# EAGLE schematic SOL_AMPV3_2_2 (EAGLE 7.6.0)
C_RIGHT: (C) 2016, 2017 Universiteit Antwerpen; D_NAME: W. Beaumont; PROJECT_NAME: SOLID AMPLIFIER; S_REV: 2.2

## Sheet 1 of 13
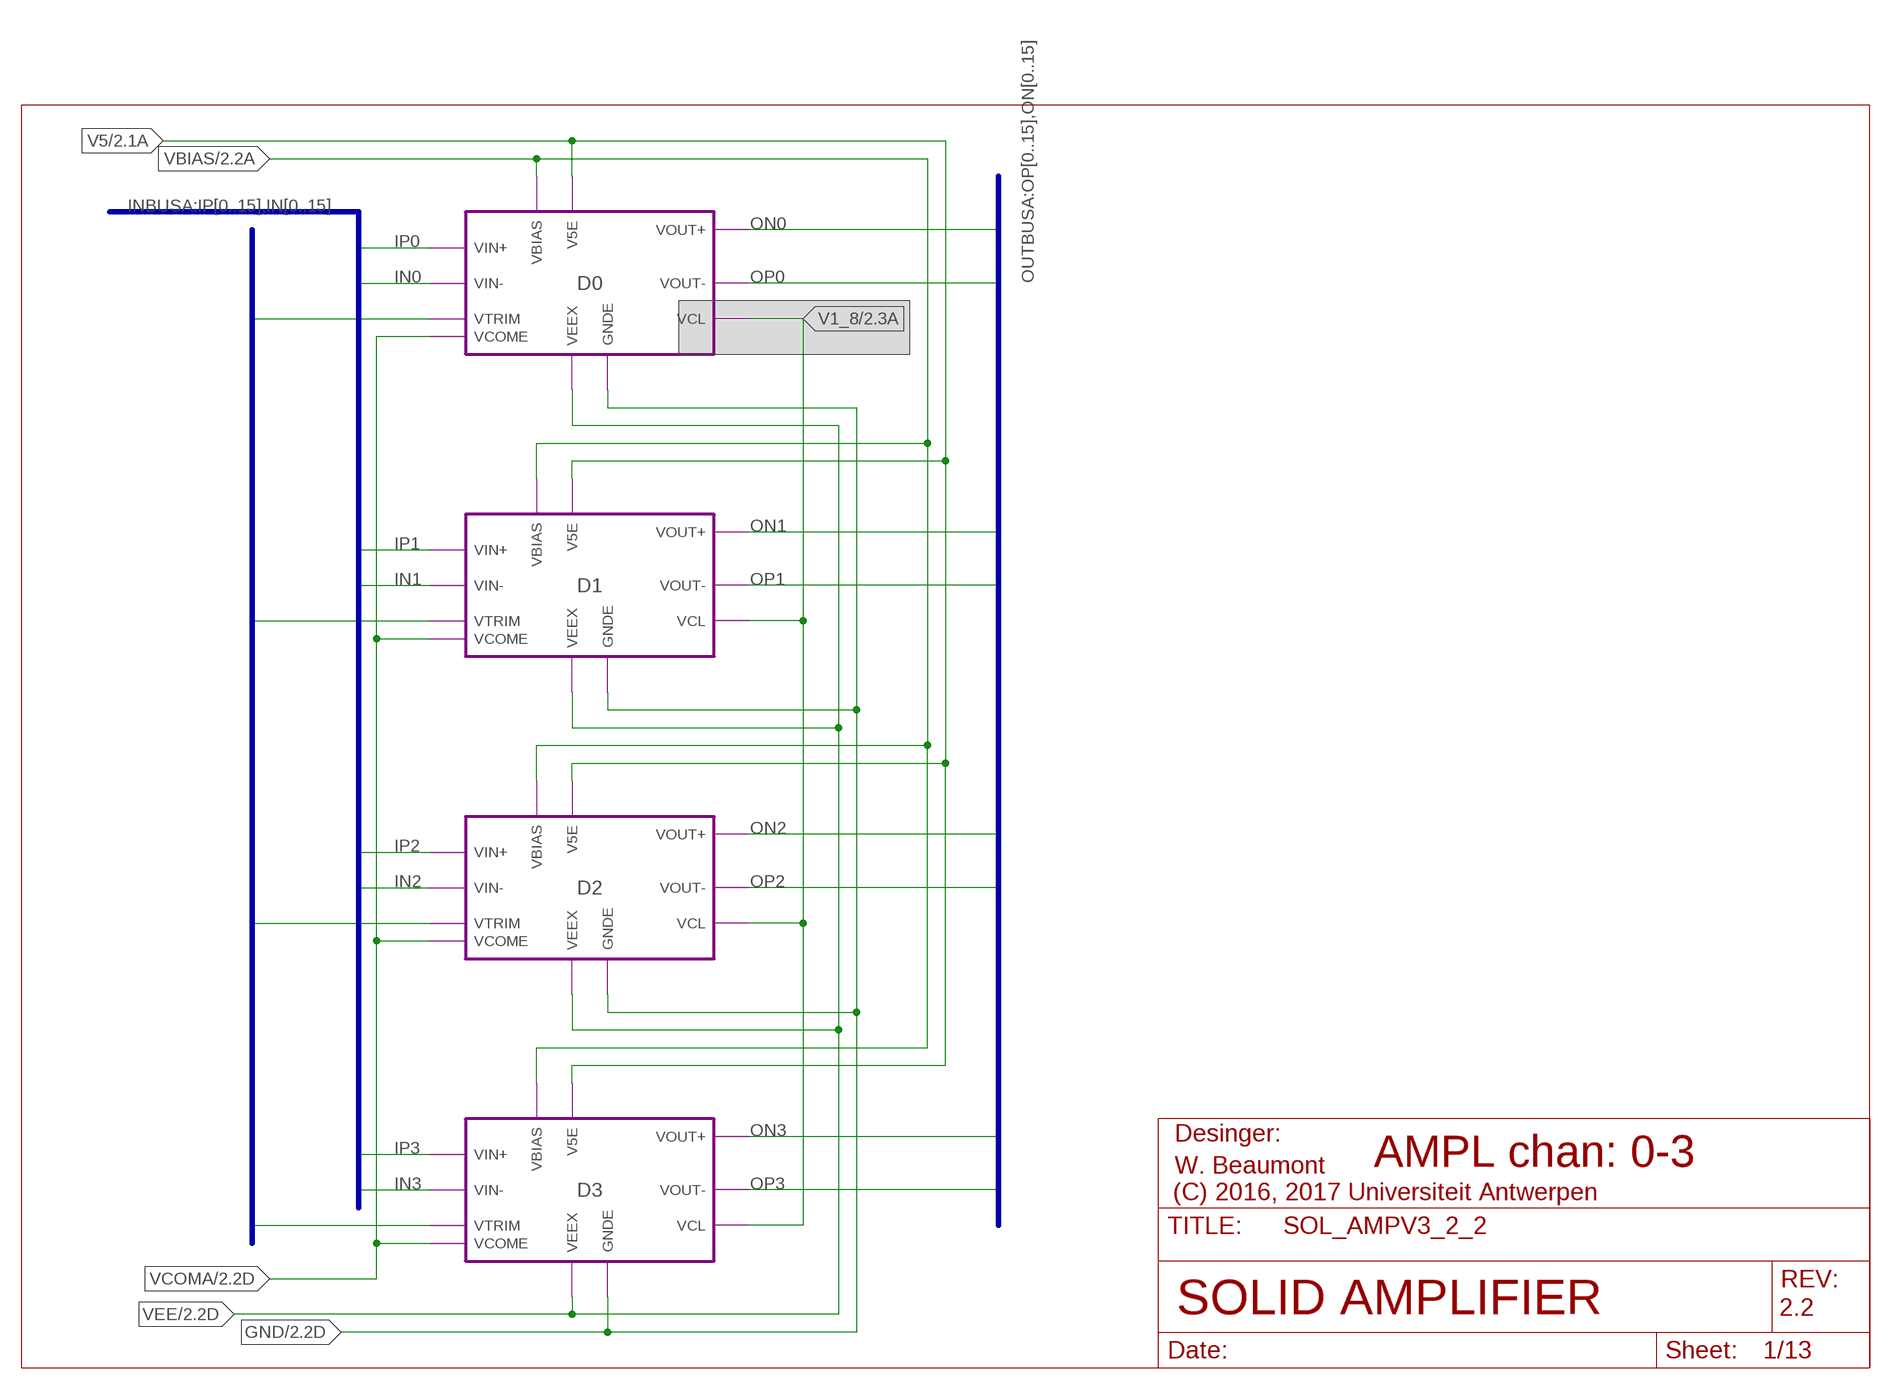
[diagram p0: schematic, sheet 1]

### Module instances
D0 = DIFFAMP$B
D1 = DIFFAMP$B
D2 = DIFFAMP$B
D3 = DIFFAMP$B

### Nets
GND: port D0.GNDE D1.GNDE D2.GNDE D3.GNDE ; also sheet 2,3,4,5,6,7,8,9,10,11,12,13
IN0: port D0.VIN- ; also sheet 5
IN1: port D1.VIN- ; also sheet 5
IN2: port D2.VIN- ; also sheet 5
IN3: port D3.VIN- ; also sheet 5
IP0: port D0.VIN+ ; also sheet 5
IP1: port D1.VIN+ ; also sheet 5
IP2: port D2.VIN+ ; also sheet 5
IP3: port D3.VIN+ ; also sheet 5
ON0: port D0.VOUT+ ; also sheet 5
ON1: port D1.VOUT+ ; also sheet 5
ON2: port D2.VOUT+ ; also sheet 5
ON3: port D3.VOUT+ ; also sheet 5
OP0: port D0.VOUT- ; also sheet 5
OP1: port D1.VOUT- ; also sheet 5
OP2: port D2.VOUT- ; also sheet 5
OP3: port D3.VOUT- ; also sheet 5
V1_8: port D3.VCL D0.VCL D1.VCL D2.VCL ; also sheet 2,3,4,5,6,7,8,9,10
V5: port D0.V5E D1.V5E D2.V5E D3.V5E ; also sheet 2,3,4,5,6,7,8,9,10,12,13
VBIAS [HV]: port D0.VBIAS D1.VBIAS D3.VBIAS D2.VBIAS ; also sheet 2,3,4,6,7,8,9,13
VCOMA: port D0.VCOME D3.VCOME D2.VCOME D1.VCOME ; also sheet 2,3,4,5
VEE: port D0.VEEX D1.VEEX D2.VEEX D3.VEEX ; also sheet 2,3,4,6,7,8,9,12
VTR0: port D0.VTRIM ; also sheet 11
VTR1: port D1.VTRIM ; also sheet 11
VTR2: port D2.VTRIM ; also sheet 11
VTR3: port D3.VTRIM ; also sheet 11

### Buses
OUTBUSA:OP[0..15],ON[0..15]
INBUSA:IP[0..15],IN[0..15]
VTRB:VTR[0..31]

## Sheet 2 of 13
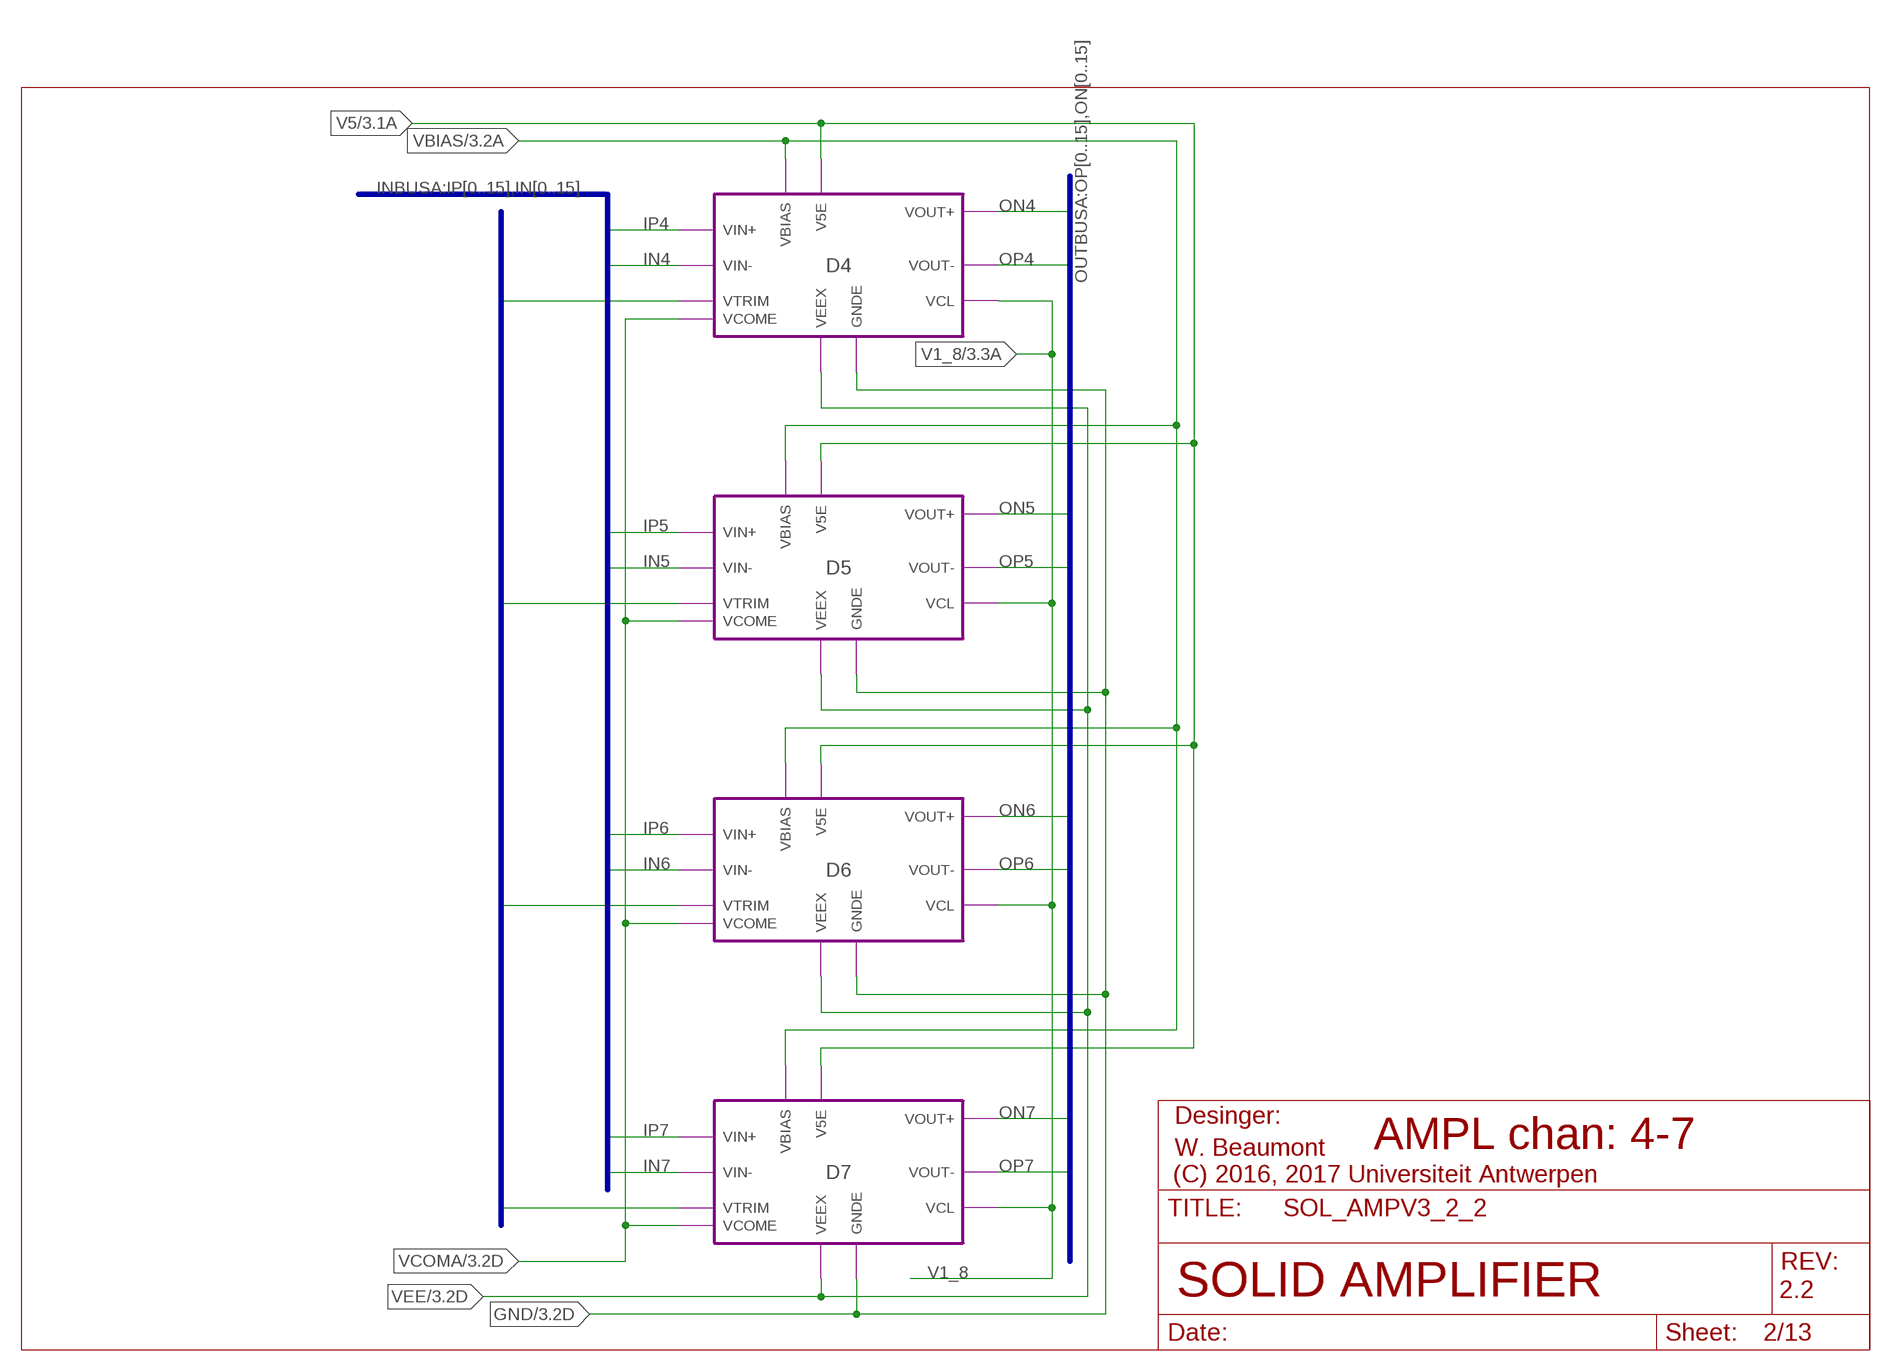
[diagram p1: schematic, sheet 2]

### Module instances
D4 = DIFFAMP$B
D5 = DIFFAMP$B
D6 = DIFFAMP$B
D7 = DIFFAMP$B

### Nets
GND: port D4.GNDE D5.GNDE D6.GNDE D7.GNDE ; also sheet 1,3,4,5,6,7,8,9,10,11,12,13
IN4: port D4.VIN- ; also sheet 5
IN5: port D5.VIN- ; also sheet 5
IN6: port D6.VIN- ; also sheet 5
IN7: port D7.VIN- ; also sheet 5
IP4: port D4.VIN+ ; also sheet 5
IP5: port D5.VIN+ ; also sheet 5
IP6: port D6.VIN+ ; also sheet 5
IP7: port D7.VIN+ ; also sheet 5
ON4: port D4.VOUT+ ; also sheet 5
ON5: port D5.VOUT+ ; also sheet 5
ON6: port D6.VOUT+ ; also sheet 5
ON7: port D7.VOUT+ ; also sheet 5
OP4: port D4.VOUT- ; also sheet 5
OP5: port D5.VOUT- ; also sheet 5
OP6: port D6.VOUT- ; also sheet 5
OP7: port D7.VOUT- ; also sheet 5
V1_8: port D4.VCL D7.VCL D6.VCL D5.VCL ; also sheet 1,3,4,5,6,7,8,9,10
V5: port D4.V5E D5.V5E D6.V5E D7.V5E ; also sheet 1,3,4,5,6,7,8,9,10,12,13
VBIAS [HV]: port D4.VBIAS D5.VBIAS D7.VBIAS D6.VBIAS ; also sheet 1,3,4,6,7,8,9,13
VCOMA: port D4.VCOME D7.VCOME D6.VCOME D5.VCOME ; also sheet 1,3,4,5
VEE: port D4.VEEX D5.VEEX D6.VEEX D7.VEEX ; also sheet 1,3,4,6,7,8,9,12
VTR4: port D4.VTRIM ; also sheet 11
VTR5: port D5.VTRIM ; also sheet 11
VTR6: port D6.VTRIM ; also sheet 11
VTR7: port D7.VTRIM ; also sheet 11

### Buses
OUTBUSA:OP[0..15],ON[0..15]
INBUSA:IP[0..15],IN[0..15]
VTRB:VTR[0..31]

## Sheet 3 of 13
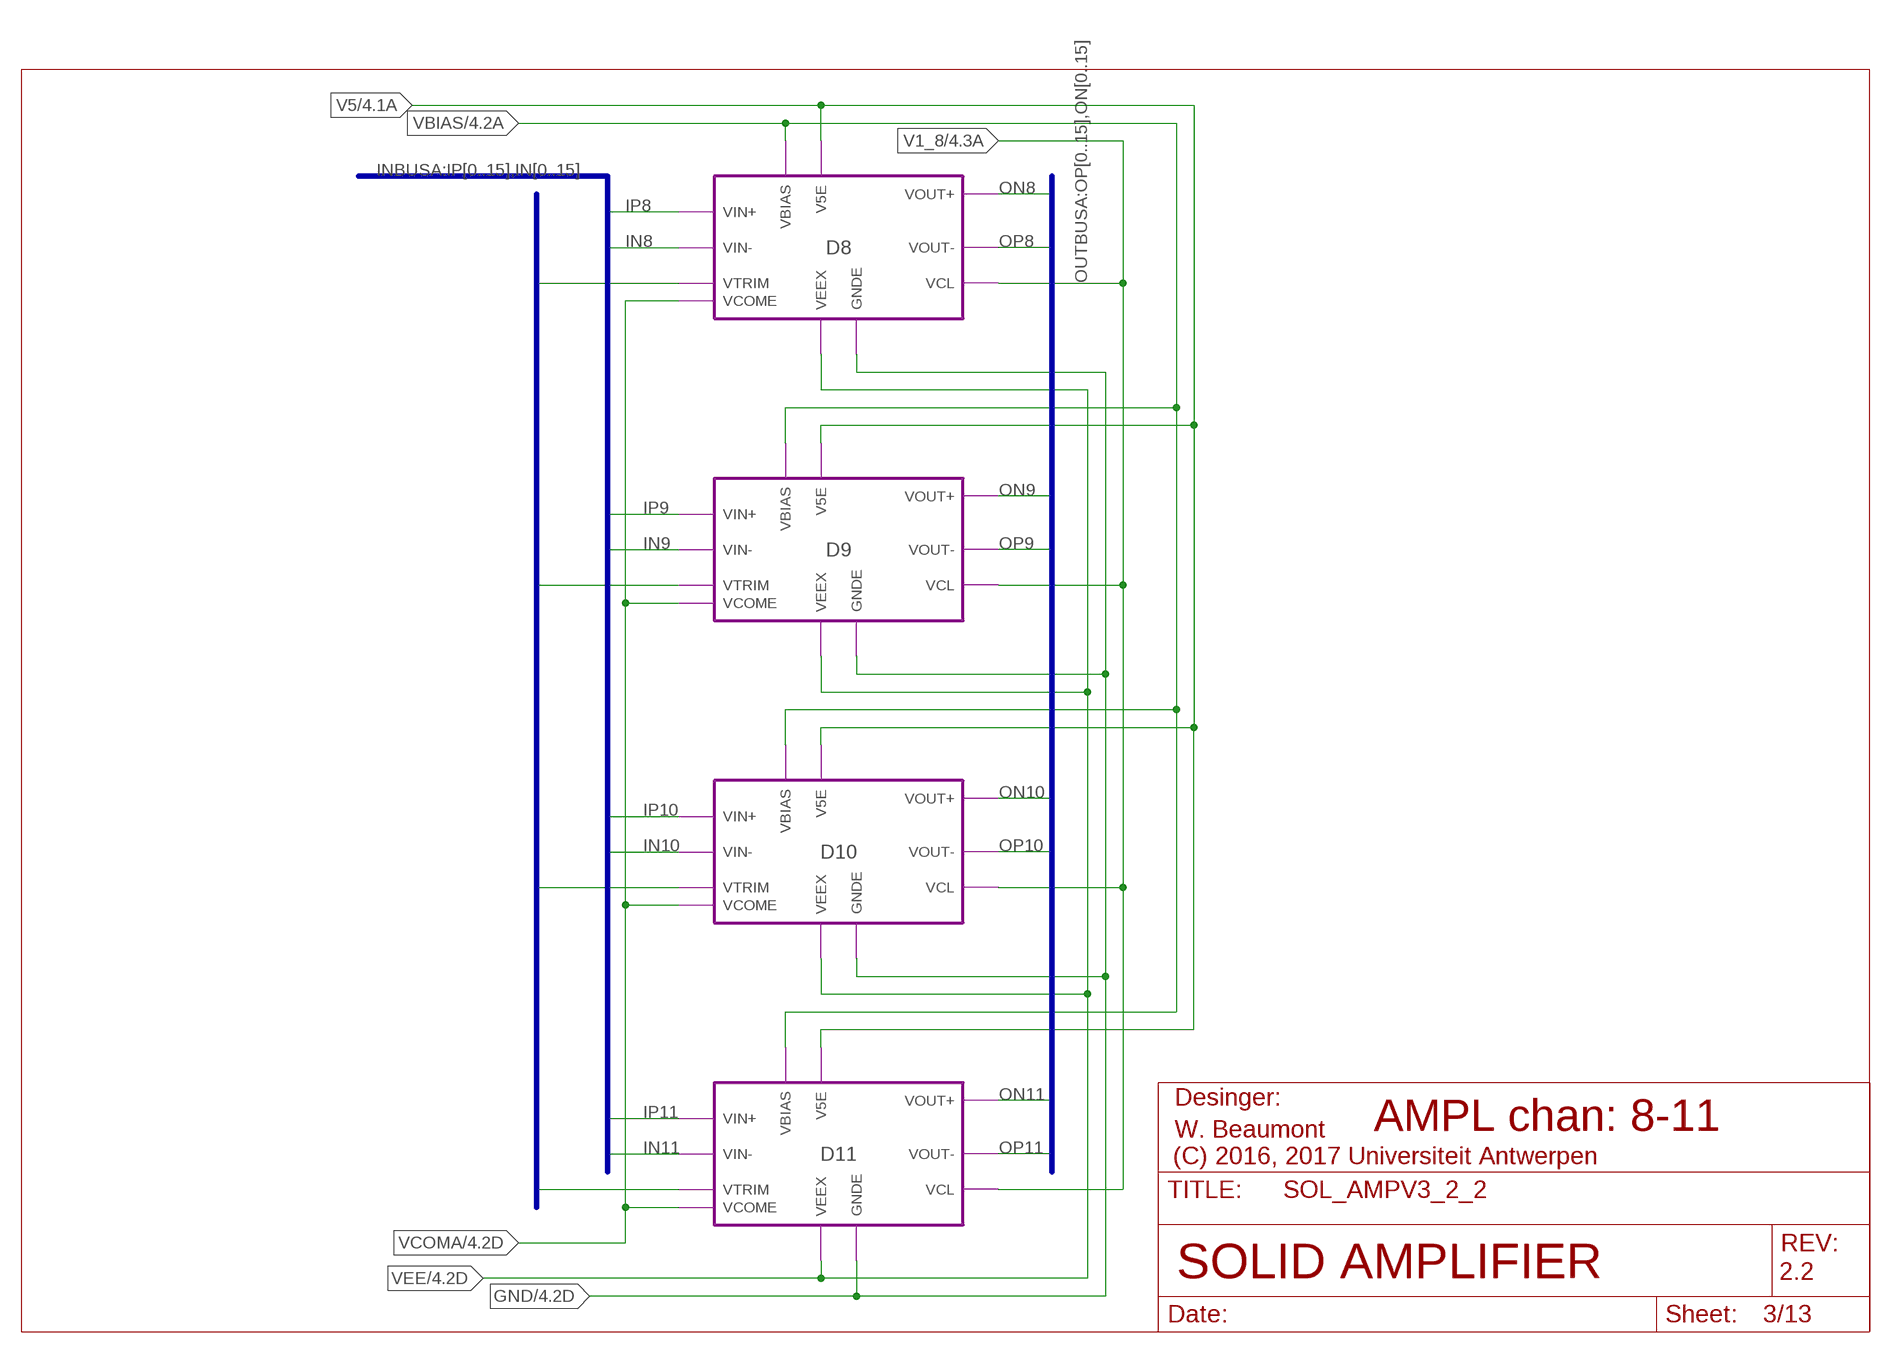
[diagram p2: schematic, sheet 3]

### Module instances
D8 = DIFFAMP$B
D9 = DIFFAMP$B
D10 = DIFFAMP$B
D11 = DIFFAMP$B

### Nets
GND: port D8.GNDE D9.GNDE D10.GNDE D11.GNDE ; also sheet 1,2,4,5,6,7,8,9,10,11,12,13
IN8: port D8.VIN- ; also sheet 5
IN9: port D9.VIN- ; also sheet 5
IN10: port D10.VIN- ; also sheet 5
IN11: port D11.VIN- ; also sheet 5
IP8: port D8.VIN+ ; also sheet 5
IP9: port D9.VIN+ ; also sheet 5
IP10: port D10.VIN+ ; also sheet 5
IP11: port D11.VIN+ ; also sheet 5
ON8: port D8.VOUT+ ; also sheet 5
ON9: port D9.VOUT+ ; also sheet 5
ON10: port D10.VOUT+ ; also sheet 5
ON11: port D11.VOUT+ ; also sheet 5
OP8: port D8.VOUT- ; also sheet 5
OP9: port D9.VOUT- ; also sheet 5
OP10: port D10.VOUT- ; also sheet 5
OP11: port D11.VOUT- ; also sheet 5
V1_8: port D11.VCL D10.VCL D9.VCL D8.VCL ; also sheet 1,2,4,5,6,7,8,9,10
V5: port D8.V5E D9.V5E D10.V5E D11.V5E ; also sheet 1,2,4,5,6,7,8,9,10,12,13
VBIAS [HV]: port D8.VBIAS D9.VBIAS D11.VBIAS D10.VBIAS ; also sheet 1,2,4,6,7,8,9,13
VCOMA: port D8.VCOME D11.VCOME D10.VCOME D9.VCOME ; also sheet 1,2,4,5
VEE: port D8.VEEX D9.VEEX D10.VEEX D11.VEEX ; also sheet 1,2,4,6,7,8,9,12
VTR8: port D8.VTRIM ; also sheet 11
VTR9: port D9.VTRIM ; also sheet 11
VTR10: port D10.VTRIM ; also sheet 11
VTR11: port D11.VTRIM ; also sheet 11

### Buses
OUTBUSA:OP[0..15],ON[0..15]
INBUSA:IP[0..15],IN[0..15]
VTRB:VTR[0..31]

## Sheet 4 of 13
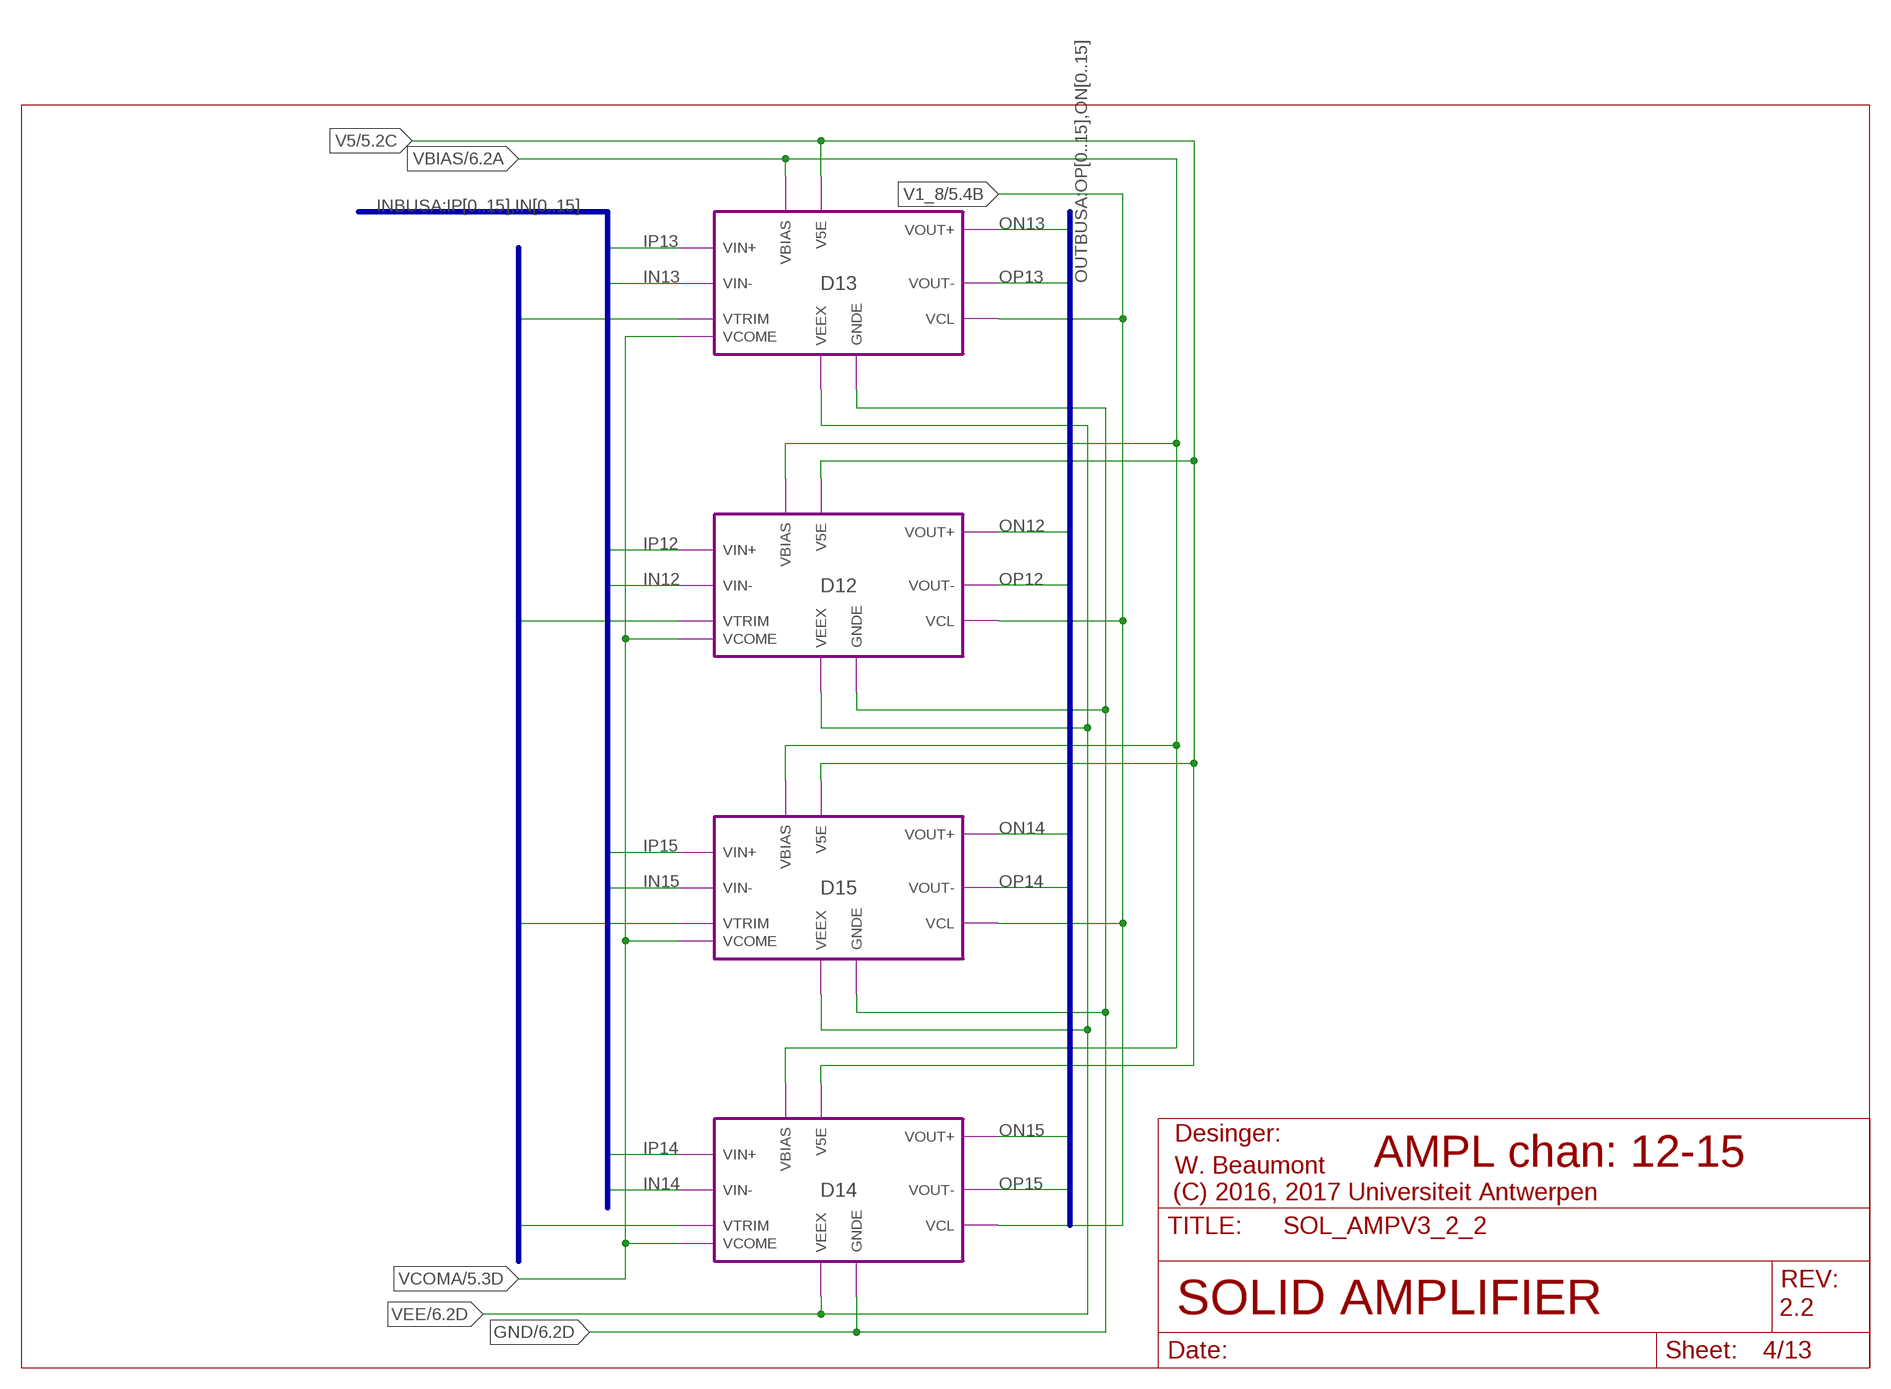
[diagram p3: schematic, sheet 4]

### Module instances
D13 = DIFFAMP$B
D12 = DIFFAMP$B
D15 = DIFFAMP$B
D14 = DIFFAMP$B

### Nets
GND: port D13.GNDE D12.GNDE D15.GNDE D14.GNDE ; also sheet 1,2,3,5,6,7,8,9,10,11,12,13
IN12: port D12.VIN- ; also sheet 5
IN13: port D13.VIN- ; also sheet 5
IN14: port D14.VIN- ; also sheet 5
IN15: port D15.VIN- ; also sheet 5
IP12: port D12.VIN+ ; also sheet 5
IP13: port D13.VIN+ ; also sheet 5
IP14: port D14.VIN+ ; also sheet 5
IP15: port D15.VIN+ ; also sheet 5
ON12: port D12.VOUT+ ; also sheet 5
ON13: port D13.VOUT+ ; also sheet 5
ON14: port D15.VOUT+ ; also sheet 5
ON15: port D14.VOUT+ ; also sheet 5
OP12: port D12.VOUT- ; also sheet 5
OP13: port D13.VOUT- ; also sheet 5
OP14: port D15.VOUT- ; also sheet 5
OP15: port D14.VOUT- ; also sheet 5
V1_8: port D13.VCL D12.VCL D15.VCL D14.VCL ; also sheet 1,2,3,5,6,7,8,9,10
V5: port D13.V5E D12.V5E D15.V5E D14.V5E ; also sheet 1,2,3,5,6,7,8,9,10,12,13
VBIAS [HV]: port D13.VBIAS D12.VBIAS D14.VBIAS D15.VBIAS ; also sheet 1,2,3,6,7,8,9,13
VCOMA: port D13.VCOME D14.VCOME D15.VCOME D12.VCOME ; also sheet 1,2,3,5
VEE: port D13.VEEX D12.VEEX D15.VEEX D14.VEEX ; also sheet 1,2,3,6,7,8,9,12
VTR12: port D13.VTRIM ; also sheet 11
VTR13: port D12.VTRIM ; also sheet 11
VTR14: port D15.VTRIM ; also sheet 11
VTR15: port D14.VTRIM ; also sheet 11

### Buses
OUTBUSA:OP[0..15],ON[0..15]
INBUSA:IP[0..15],IN[0..15]
VTRB:VTR[0..31]

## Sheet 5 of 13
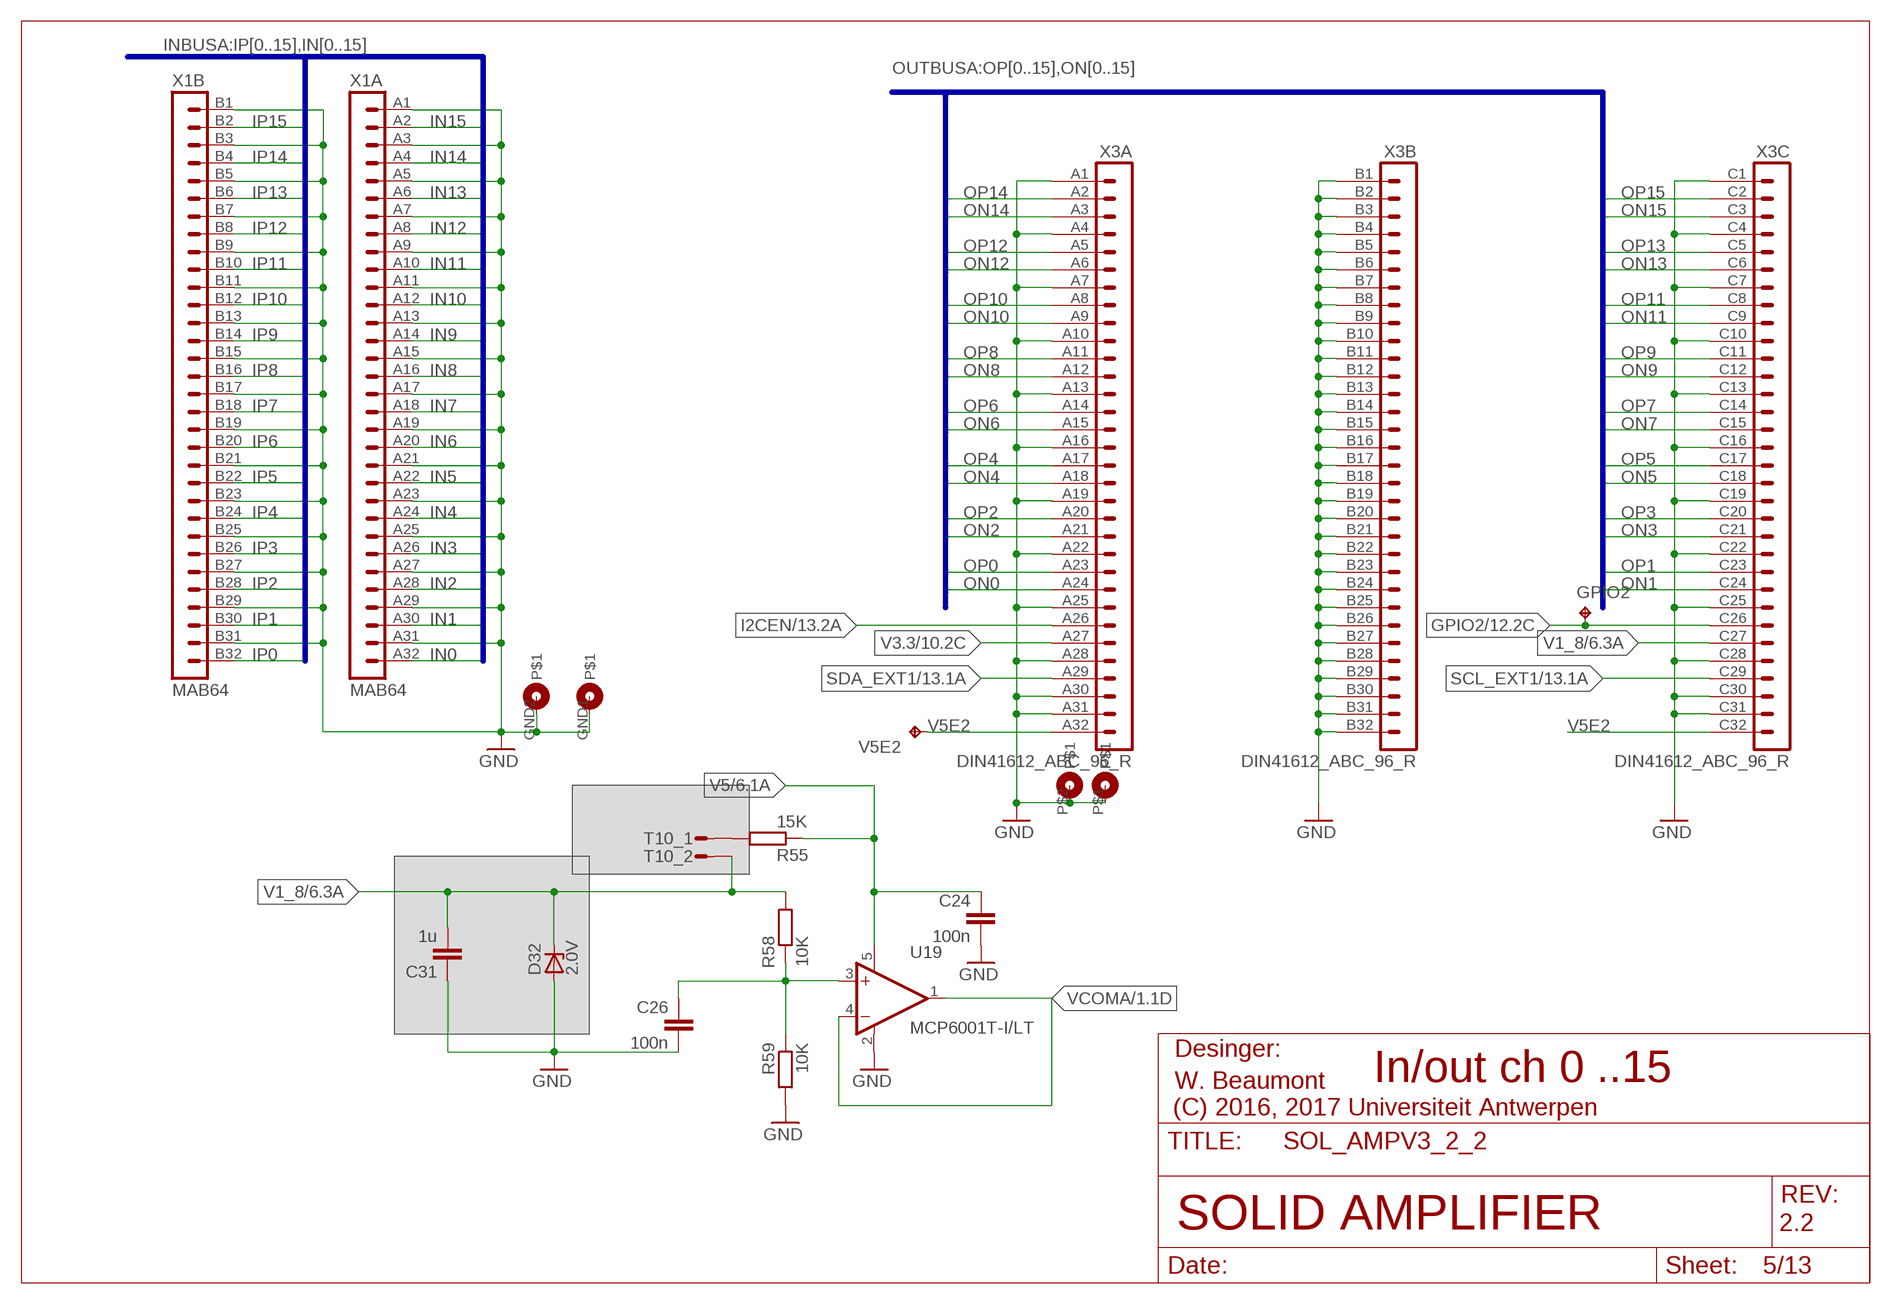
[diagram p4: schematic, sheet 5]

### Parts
C24  100n  C-EUC0402  [C0402]
C26  100n  C-EUC0402  [C0402]
C31  1u  C-EUC0402  [C0402]
D32  2.0V  TFZV  [SOD323R_ROHM]
GPIO2  UA_TPPAD1-13  [UA_P1-13]
R55  15K  R-EU_R0402  [R0402]
R58  10K  R-EU_R0402  [R0402]
R59  10K  R-EU_R0402  [R0402]
T10  nc  UATP1X2  [UATP1X2]
U19  MCP6001T-I/LT  [SOT65P240X110-5N]
V5E2  UA_TPPAD1-13  [UA_P1-13]
X1  MAB64  [MAB64]
X3  DIN41612_ABC_96_R  [DIN41612_96RC]

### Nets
GND: C24.2 C26.2 C31.1 D32.A R59.2 U19.2(V-) X1.A1 X1.A3 X1.A5 X1.A7 X1.A9 X1.A11 X1.A13 X1.A15 X1.A17 X1.A19 X1.A21 X1.A23 X1.A25 X1.A27 X1.A29 X1.A31 X1.B1 X1.B3 X1.B5 X1.B7 X1.B9 X1.B11 X1.B13 X1.B15 X1.B17 X1.B19 X1.B21 X1.B23 X1.B25 X1.B27 X1.B29 X1.B31 X1.GND1 X1.GND2 X3.A1 X3.A4 X3.A7 X3.A10 X3.A13 X3.A16 X3.A19 X3.A22 X3.A25 X3.A28 X3.A30 X3.A31 X3.B1 X3.B2 X3.B3 X3.B4 X3.B5 X3.B6 X3.B7 X3.B8 X3.B9 X3.B10 X3.B11 X3.B12 X3.B13 X3.B14 X3.B15 X3.B16 X3.B17 X3.B18 X3.B19 X3.B20 X3.B21 X3.B22 X3.B23 X3.B24 X3.B25 X3.B26 X3.B27 X3.B28 X3.B29 X3.B30 X3.B31 X3.B32 X3.C1 X3.C4 X3.C7 X3.C10 X3.C13 X3.C16 X3.C19 X3.C22 X3.C25 X3.C28 X3.C30 X3.C31 X3.P$1 X3.P$2 ; also sheet 1,2,3,4,6,7,8,9,10,11,12,13
GPIO2: GPIO2.TP X3.C26 ; also sheet 12
I2CEN: X3.A26 ; also sheet 13
IN0: X1.A32 ; also sheet 1
IN1: X1.A30 ; also sheet 1
IN2: X1.A28 ; also sheet 1
IN3: X1.A26 ; also sheet 1
IN4: X1.A24 ; also sheet 2
IN5: X1.A22 ; also sheet 2
IN6: X1.A20 ; also sheet 2
IN7: X1.A18 ; also sheet 2
IN8: X1.A16 ; also sheet 3
IN9: X1.A14 ; also sheet 3
IN10: X1.A12 ; also sheet 3
IN11: X1.A10 ; also sheet 3
IN12: X1.A8 ; also sheet 4
IN13: X1.A6 ; also sheet 4
IN14: X1.A4 ; also sheet 4
IN15: X1.A2 ; also sheet 4
IP0: X1.B32 ; also sheet 1
IP1: X1.B30 ; also sheet 1
IP2: X1.B28 ; also sheet 1
IP3: X1.B26 ; also sheet 1
IP4: X1.B24 ; also sheet 2
IP5: X1.B22 ; also sheet 2
IP6: X1.B20 ; also sheet 2
IP7: X1.B18 ; also sheet 2
IP8: X1.B16 ; also sheet 3
IP9: X1.B14 ; also sheet 3
IP10: X1.B12 ; also sheet 3
IP11: X1.B10 ; also sheet 3
IP12: X1.B8 ; also sheet 4
IP13: X1.B6 ; also sheet 4
IP14: X1.B4 ; also sheet 4
IP15: X1.B2 ; also sheet 4
N$23: C26.1 R58.2 R59.1 U19.3(+IN)
N$28: R55.1 T10.1
ON0: X3.A24 ; also sheet 1
ON1: X3.C24 ; also sheet 1
ON2: X3.A21 ; also sheet 1
ON3: X3.C21 ; also sheet 1
ON4: X3.A18 ; also sheet 2
ON5: X3.C18 ; also sheet 2
ON6: X3.A15 ; also sheet 2
ON7: X3.C15 ; also sheet 2
ON8: X3.A12 ; also sheet 3
ON9: X3.C12 ; also sheet 3
ON10: X3.A9 ; also sheet 3
ON11: X3.C9 ; also sheet 3
ON12: X3.A6 ; also sheet 4
ON13: X3.C6 ; also sheet 4
ON14: X3.A3 ; also sheet 4
ON15: X3.C3 ; also sheet 4
OP0: X3.A23 ; also sheet 1
OP1: X3.C23 ; also sheet 1
OP2: X3.A20 ; also sheet 1
OP3: X3.C20 ; also sheet 1
OP4: X3.A17 ; also sheet 2
OP5: X3.C17 ; also sheet 2
OP6: X3.A14 ; also sheet 2
OP7: X3.C14 ; also sheet 2
OP8: X3.A11 ; also sheet 3
OP9: X3.C11 ; also sheet 3
OP10: X3.A8 ; also sheet 3
OP11: X3.C8 ; also sheet 3
OP12: X3.A5 ; also sheet 4
OP13: X3.C5 ; also sheet 4
OP14: X3.A2 ; also sheet 4
OP15: X3.C2 ; also sheet 4
SCL_EXT1: X3.C29 ; also sheet 13
SDA_EXT1: X3.A29 ; also sheet 13
V1_8: C31.2 D32.C R58.1 T10.2 X3.C27 ; also sheet 1,2,3,4,6,7,8,9,10
V3.3: X3.A27 ; also sheet 10,13
V5: C24.1 R55.2 U19.5(V+) ; also sheet 1,2,3,4,6,7,8,9,10,12,13
V5E2: V5E2.TP X3.A32 X3.C32
VCOMA: U19.1(OUT) U19.4(-IN) ; also sheet 1,2,3,4

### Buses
OUTBUSA:OP[0..15],ON[0..15]
INBUSA:IP[0..15],IN[0..15]

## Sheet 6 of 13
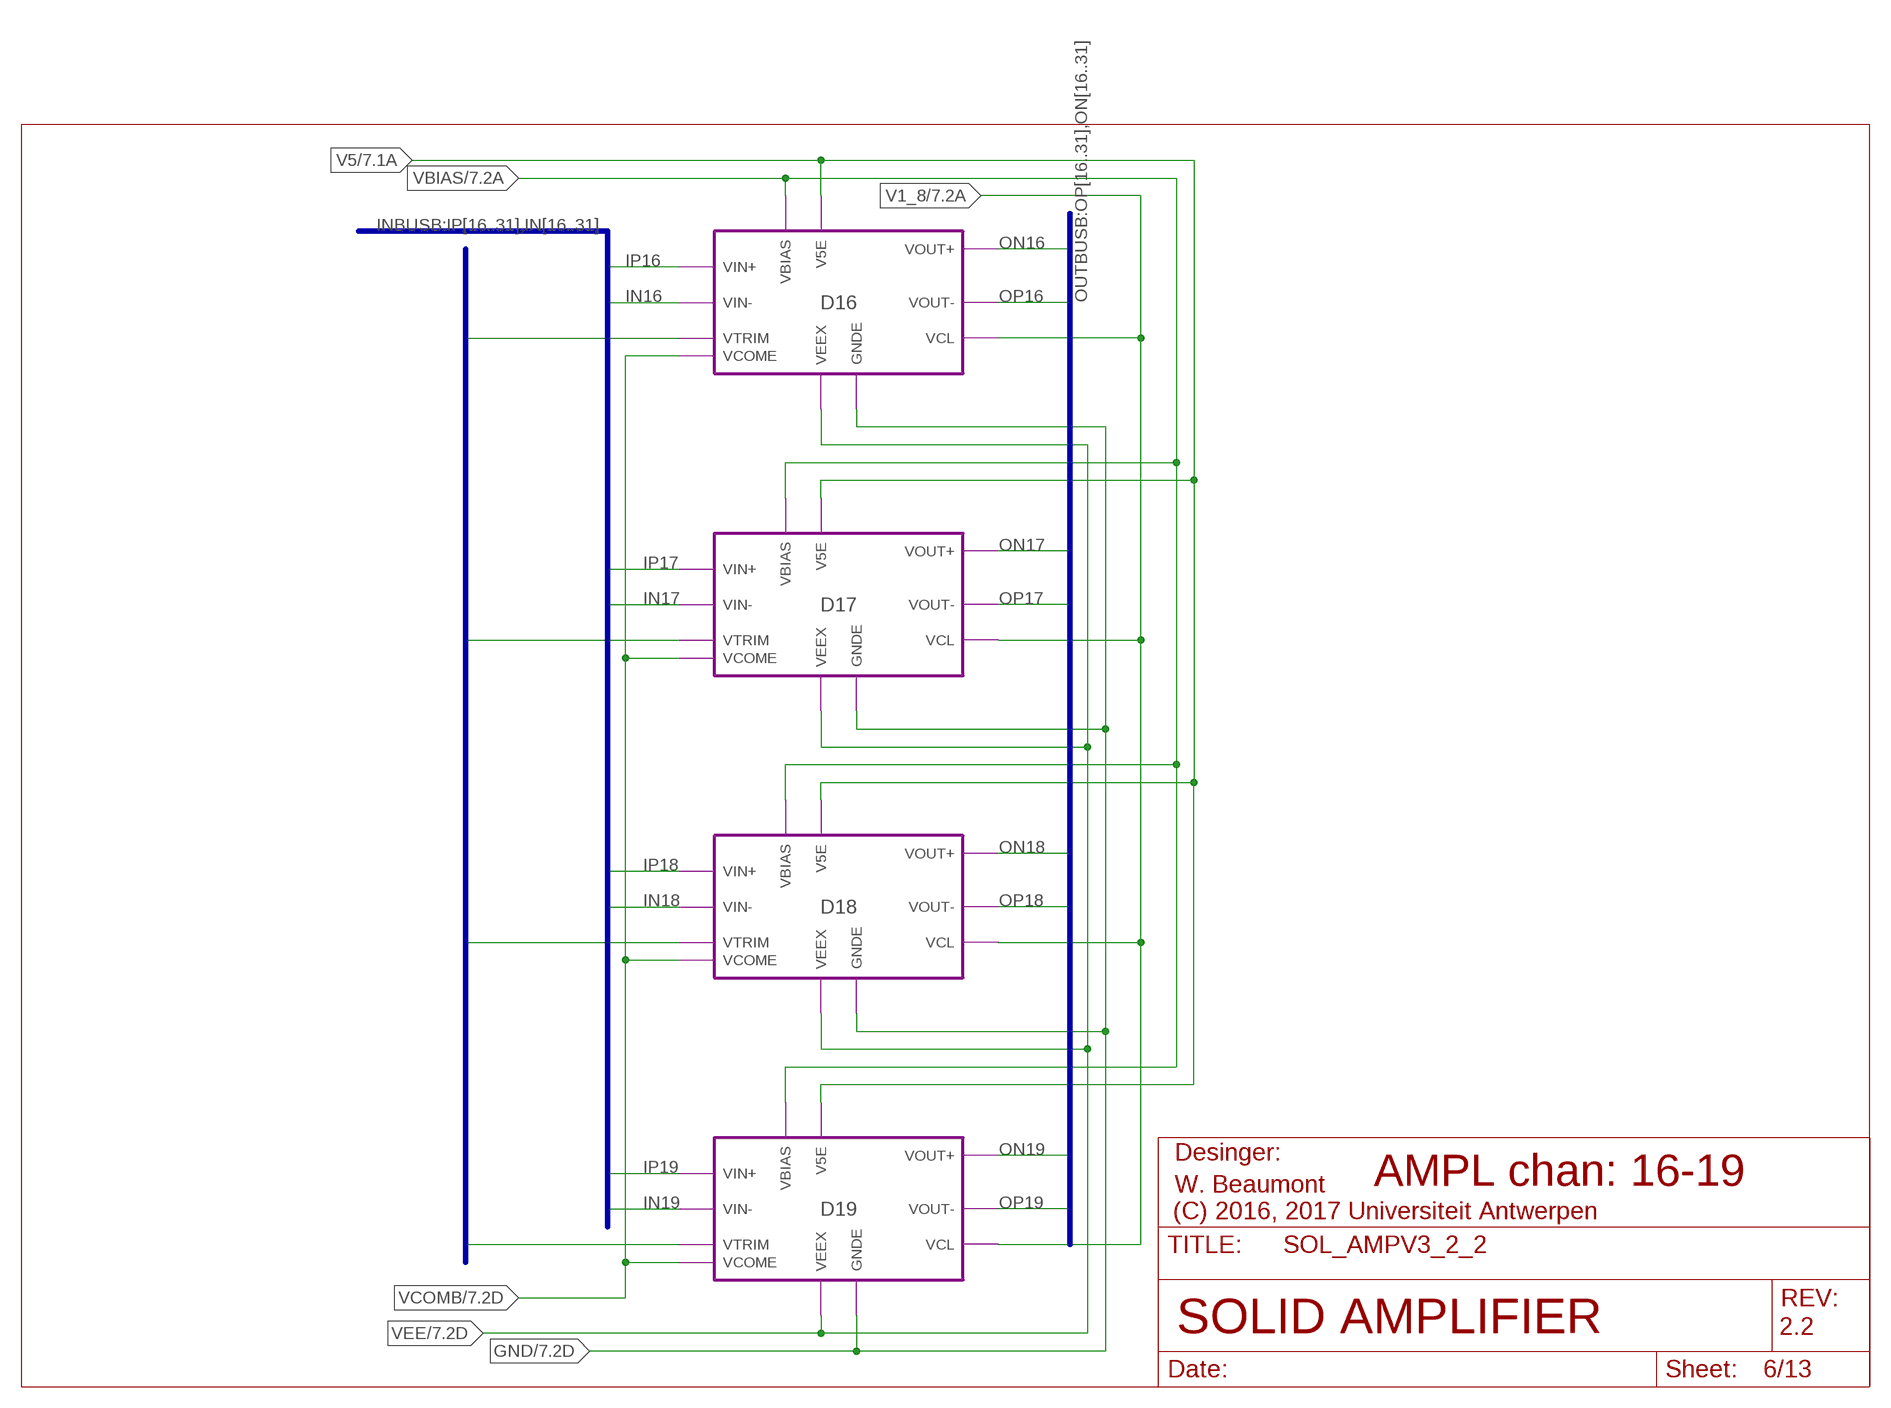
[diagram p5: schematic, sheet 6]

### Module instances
D16 = DIFFAMP$B
D17 = DIFFAMP$B
D18 = DIFFAMP$B
D19 = DIFFAMP$B

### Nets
GND: port D16.GNDE D17.GNDE D18.GNDE D19.GNDE ; also sheet 1,2,3,4,5,7,8,9,10,11,12,13
IN16: port D16.VIN- ; also sheet 10
IN17: port D17.VIN- ; also sheet 10
IN18: port D18.VIN- ; also sheet 10
IN19: port D19.VIN- ; also sheet 10
IP16: port D16.VIN+ ; also sheet 10
IP17: port D17.VIN+ ; also sheet 10
IP18: port D18.VIN+ ; also sheet 10
IP19: port D19.VIN+ ; also sheet 10
ON16: port D16.VOUT+ ; also sheet 10
ON17: port D17.VOUT+ ; also sheet 10
ON18: port D18.VOUT+ ; also sheet 10
ON19: port D19.VOUT+ ; also sheet 10
OP16: port D16.VOUT- ; also sheet 10
OP17: port D17.VOUT- ; also sheet 10
OP18: port D18.VOUT- ; also sheet 10
OP19: port D19.VOUT- ; also sheet 10
V1_8: port D19.VCL D16.VCL D17.VCL D18.VCL ; also sheet 1,2,3,4,5,7,8,9,10
V5: port D16.V5E D17.V5E D18.V5E D19.V5E ; also sheet 1,2,3,4,5,7,8,9,10,12,13
VBIAS [HV]: port D16.VBIAS D17.VBIAS D19.VBIAS D18.VBIAS ; also sheet 1,2,3,4,7,8,9,13
VCOMB: port D16.VCOME D19.VCOME D18.VCOME D17.VCOME ; also sheet 7,8,9,10
VEE: port D16.VEEX D17.VEEX D18.VEEX D19.VEEX ; also sheet 1,2,3,4,7,8,9,12
VTR16: port D16.VTRIM ; also sheet 11
VTR17: port D17.VTRIM ; also sheet 11
VTR18: port D18.VTRIM ; also sheet 11
VTR19: port D19.VTRIM ; also sheet 11

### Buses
OUTBUSB:OP[16..31],ON[16..31]
INBUSB:IP[16..31],IN[16..31]
VTRB:VTR[0..31]

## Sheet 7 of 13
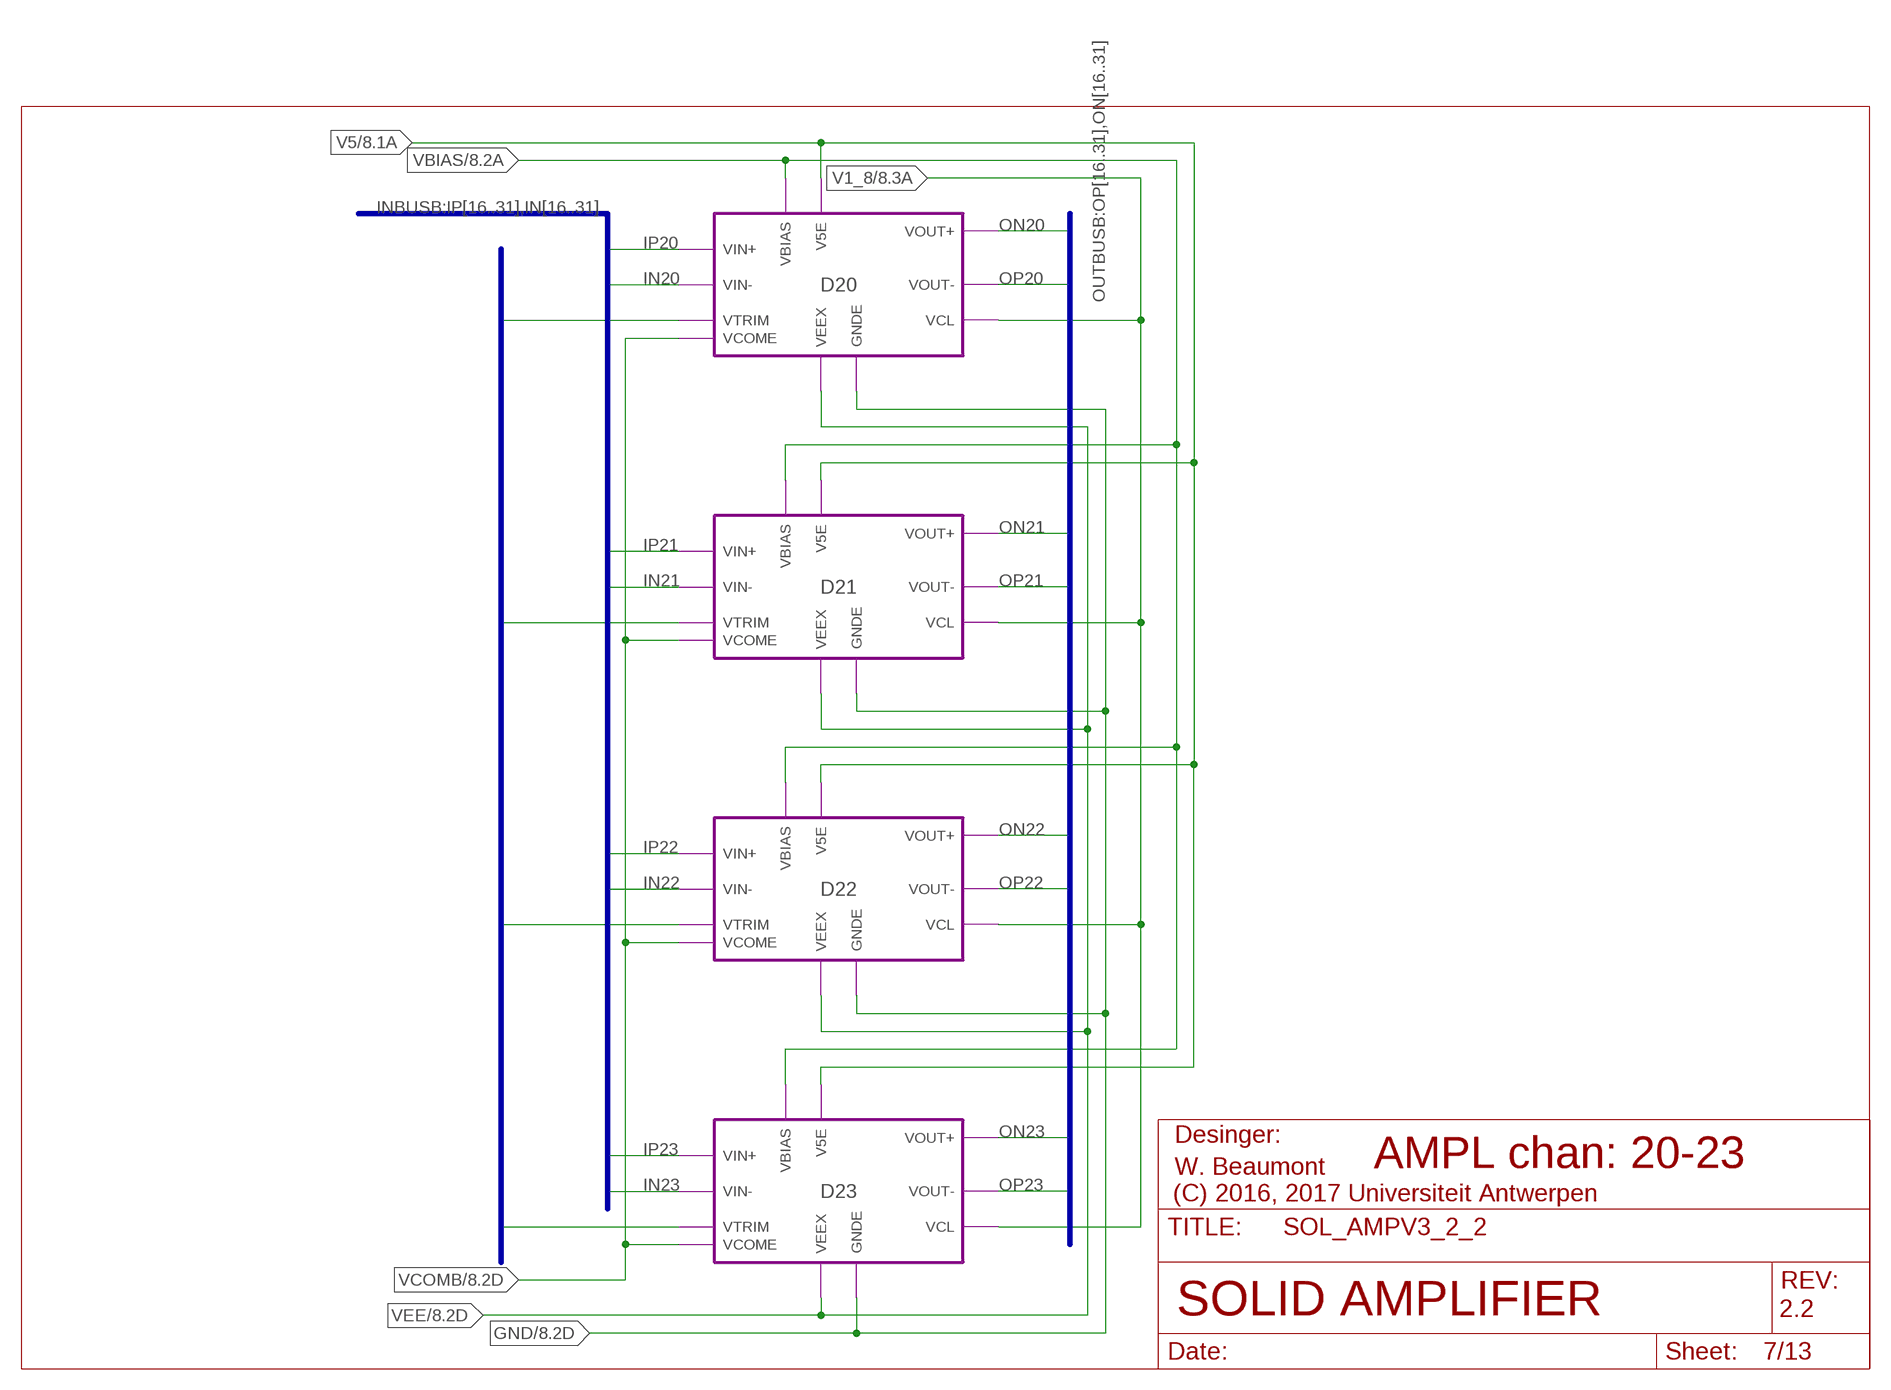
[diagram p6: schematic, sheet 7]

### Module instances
D20 = DIFFAMP$B
D21 = DIFFAMP$B
D22 = DIFFAMP$B
D23 = DIFFAMP$B

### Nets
GND: port D20.GNDE D21.GNDE D22.GNDE D23.GNDE ; also sheet 1,2,3,4,5,6,8,9,10,11,12,13
IN20: port D20.VIN- ; also sheet 10
IN21: port D21.VIN- ; also sheet 10
IN22: port D22.VIN- ; also sheet 10
IN23: port D23.VIN- ; also sheet 10
IP20: port D20.VIN+ ; also sheet 10
IP21: port D21.VIN+ ; also sheet 10
IP22: port D22.VIN+ ; also sheet 10
IP23: port D23.VIN+ ; also sheet 10
ON20: port D20.VOUT+ ; also sheet 10
ON21: port D21.VOUT+ ; also sheet 10
ON22: port D22.VOUT+ ; also sheet 10
ON23: port D23.VOUT+ ; also sheet 10
OP20: port D20.VOUT- ; also sheet 10
OP21: port D21.VOUT- ; also sheet 10
OP22: port D22.VOUT- ; also sheet 10
OP23: port D23.VOUT- ; also sheet 10
V1_8: port D23.VCL D20.VCL D21.VCL D22.VCL ; also sheet 1,2,3,4,5,6,8,9,10
V5: port D20.V5E D21.V5E D22.V5E D23.V5E ; also sheet 1,2,3,4,5,6,8,9,10,12,13
VBIAS [HV]: port D20.VBIAS D21.VBIAS D23.VBIAS D22.VBIAS ; also sheet 1,2,3,4,6,8,9,13
VCOMB: port D20.VCOME D23.VCOME D22.VCOME D21.VCOME ; also sheet 6,8,9,10
VEE: port D20.VEEX D21.VEEX D22.VEEX D23.VEEX ; also sheet 1,2,3,4,6,8,9,12
VTR20: port D20.VTRIM ; also sheet 11
VTR21: port D21.VTRIM ; also sheet 11
VTR22: port D22.VTRIM ; also sheet 11
VTR23: port D23.VTRIM ; also sheet 11

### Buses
OUTBUSB:OP[16..31],ON[16..31]
INBUSB:IP[16..31],IN[16..31]
VTRB:VTR[0..31]

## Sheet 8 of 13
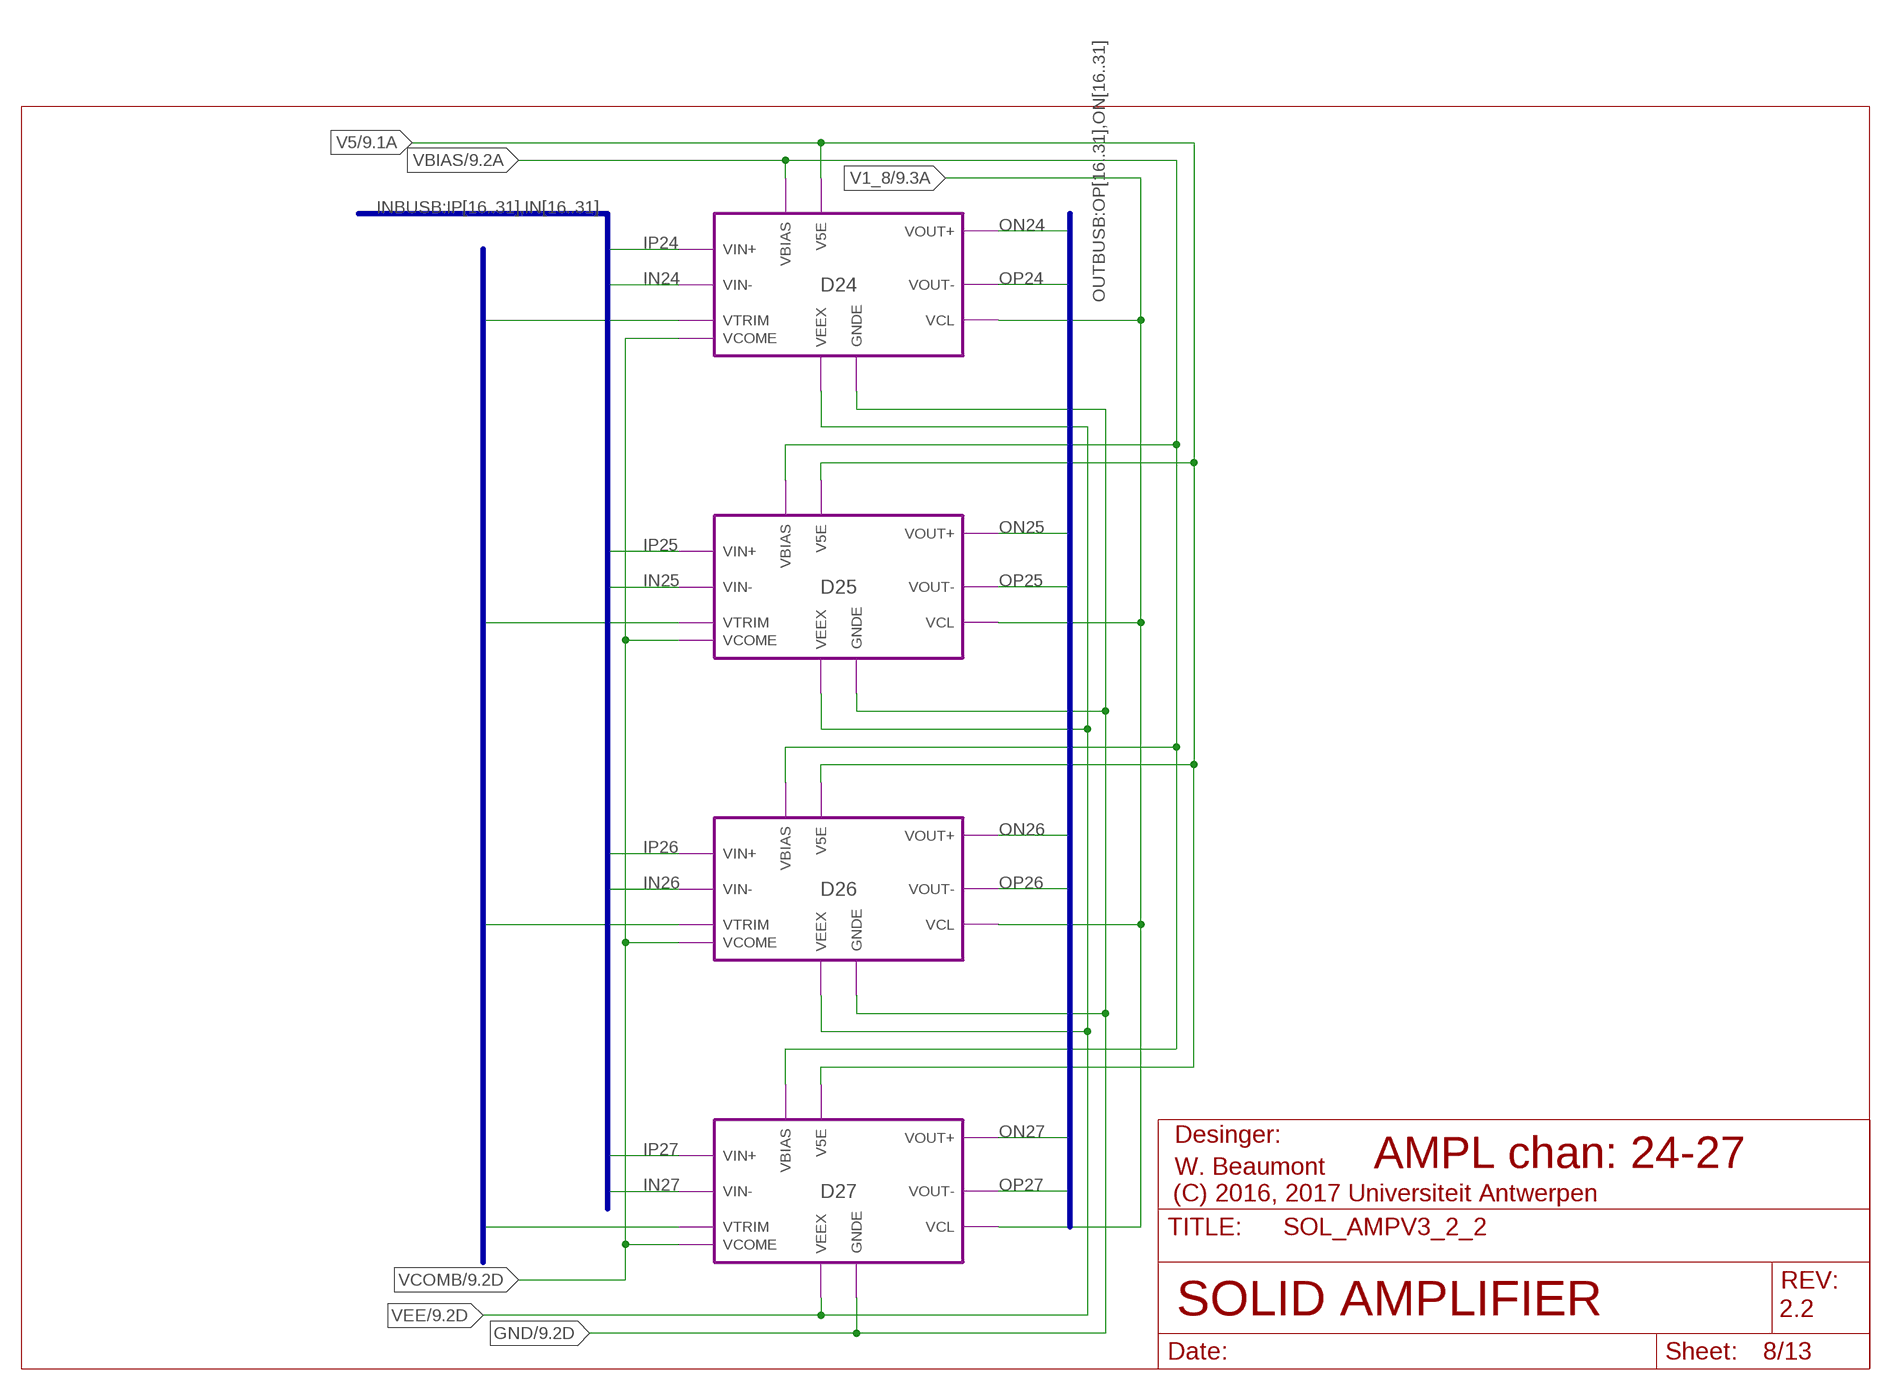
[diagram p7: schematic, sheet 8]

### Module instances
D24 = DIFFAMP$B
D25 = DIFFAMP$B
D26 = DIFFAMP$B
D27 = DIFFAMP$B

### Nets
GND: port D24.GNDE D25.GNDE D26.GNDE D27.GNDE ; also sheet 1,2,3,4,5,6,7,9,10,11,12,13
IN24: port D24.VIN- ; also sheet 10
IN25: port D25.VIN- ; also sheet 10
IN26: port D26.VIN- ; also sheet 10
IN27: port D27.VIN- ; also sheet 10
IP24: port D24.VIN+ ; also sheet 10
IP25: port D25.VIN+ ; also sheet 10
IP26: port D26.VIN+ ; also sheet 10
IP27: port D27.VIN+ ; also sheet 10
ON24: port D24.VOUT+ ; also sheet 10
ON25: port D25.VOUT+ ; also sheet 10
ON26: port D26.VOUT+ ; also sheet 10
ON27: port D27.VOUT+ ; also sheet 10
OP24: port D24.VOUT- ; also sheet 10
OP25: port D25.VOUT- ; also sheet 10
OP26: port D26.VOUT- ; also sheet 10
OP27: port D27.VOUT- ; also sheet 10
V1_8: port D27.VCL D24.VCL D26.VCL D25.VCL ; also sheet 1,2,3,4,5,6,7,9,10
V5: port D24.V5E D25.V5E D26.V5E D27.V5E ; also sheet 1,2,3,4,5,6,7,9,10,12,13
VBIAS [HV]: port D24.VBIAS D25.VBIAS D27.VBIAS D26.VBIAS ; also sheet 1,2,3,4,6,7,9,13
VCOMB: port D24.VCOME D27.VCOME D26.VCOME D25.VCOME ; also sheet 6,7,9,10
VEE: port D24.VEEX D25.VEEX D26.VEEX D27.VEEX ; also sheet 1,2,3,4,6,7,9,12
VTR24: port D24.VTRIM ; also sheet 11
VTR25: port D25.VTRIM ; also sheet 11
VTR26: port D26.VTRIM ; also sheet 11
VTR27: port D27.VTRIM ; also sheet 11

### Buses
OUTBUSB:OP[16..31],ON[16..31]
INBUSB:IP[16..31],IN[16..31]
VTRB:VTR[0..31]

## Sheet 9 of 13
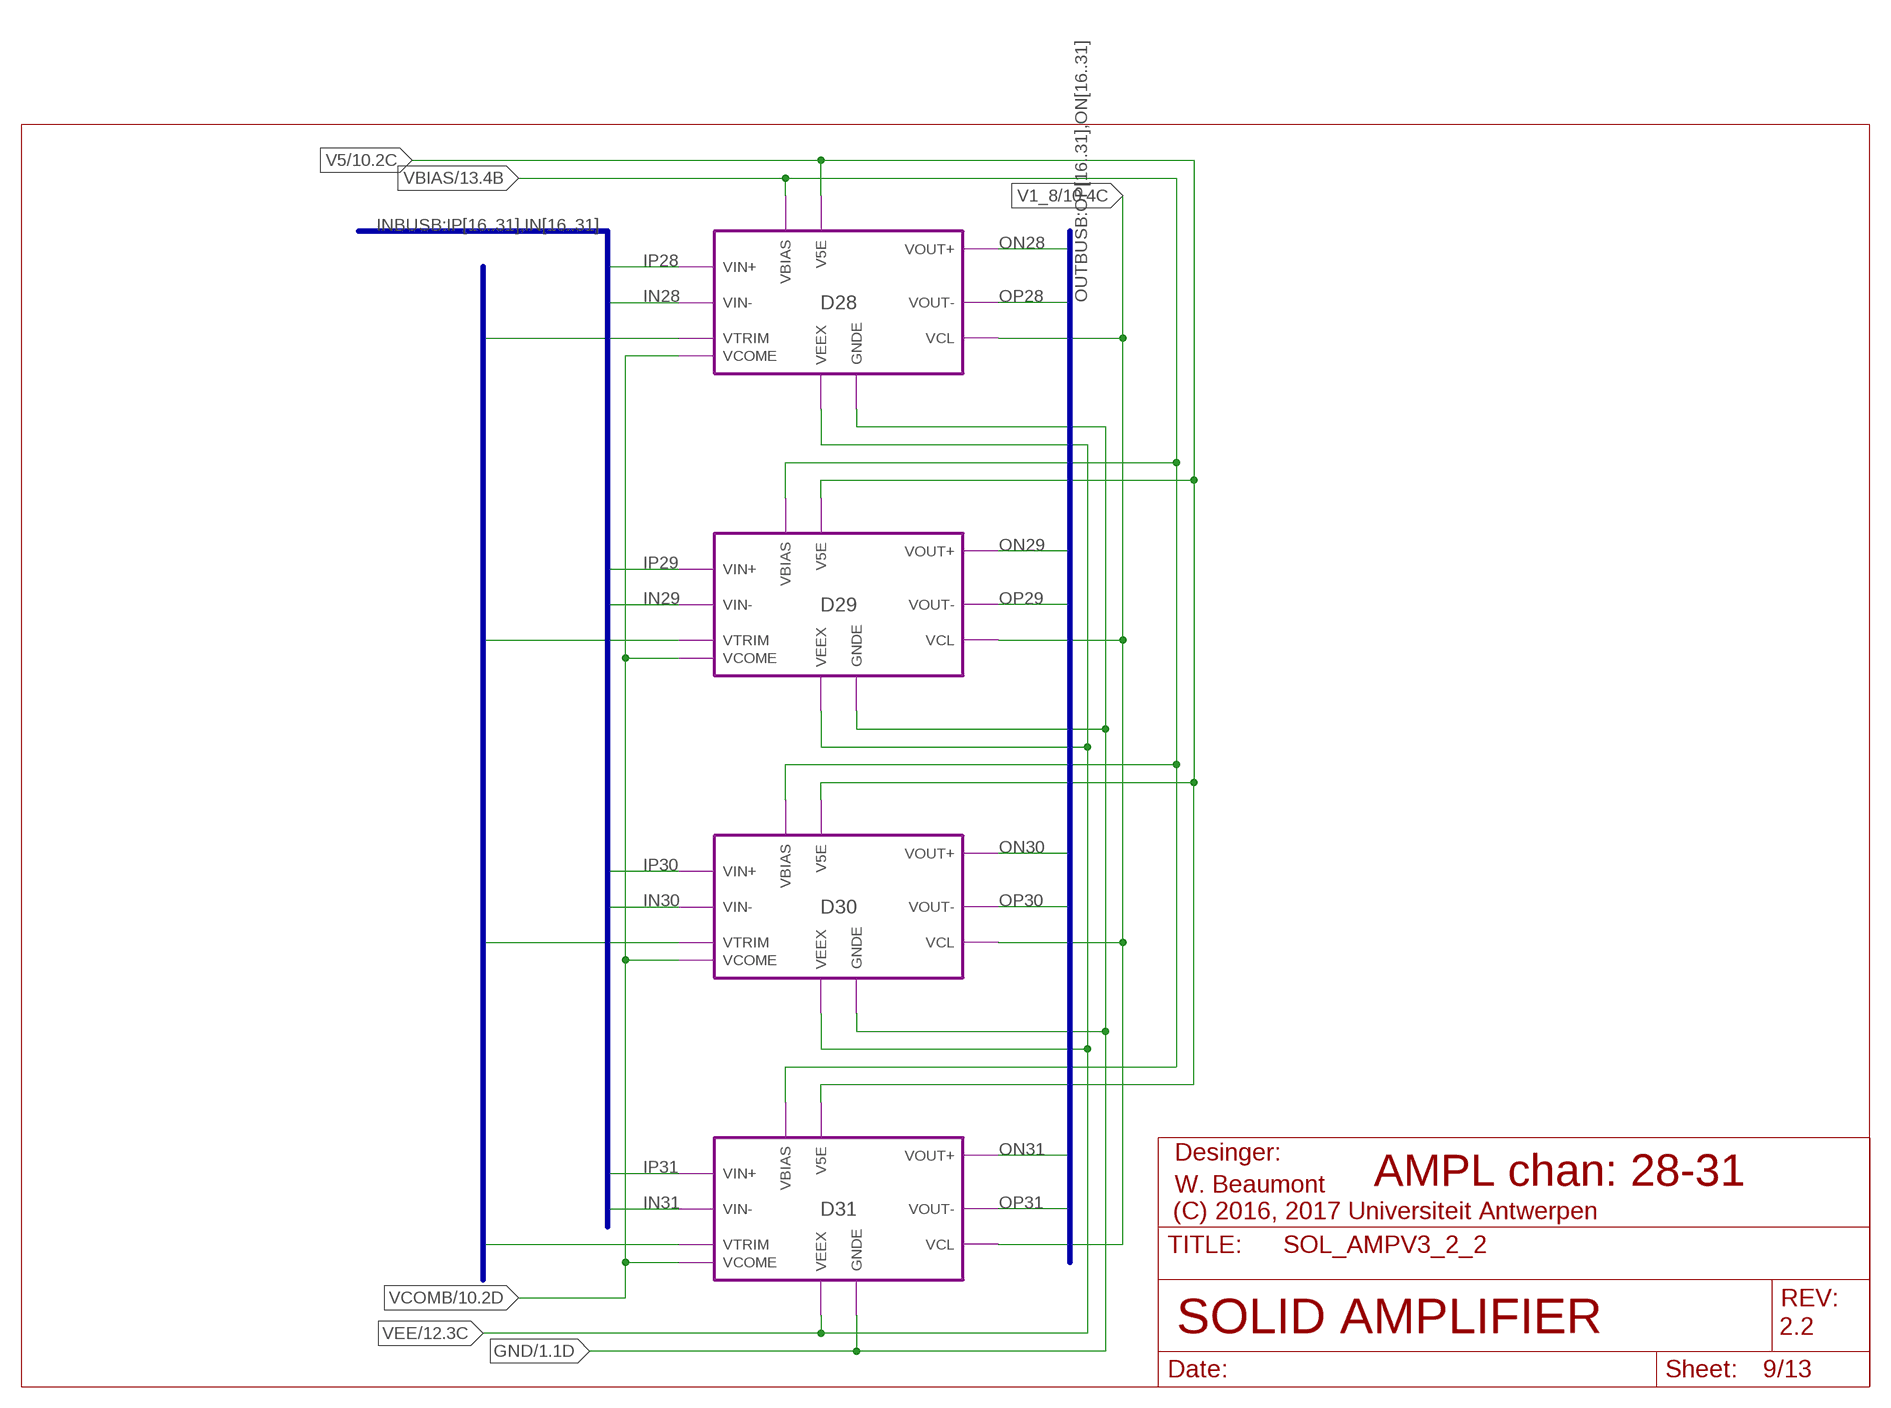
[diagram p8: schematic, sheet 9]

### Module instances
D28 = DIFFAMP$B
D29 = DIFFAMP$B
D30 = DIFFAMP$B
D31 = DIFFAMP$B

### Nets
GND: port D28.GNDE D29.GNDE D30.GNDE D31.GNDE ; also sheet 1,2,3,4,5,6,7,8,10,11,12,13
IN28: port D28.VIN- ; also sheet 10
IN29: port D29.VIN- ; also sheet 10
IN30: port D30.VIN- ; also sheet 10
IN31: port D31.VIN- ; also sheet 10
IP28: port D28.VIN+ ; also sheet 10
IP29: port D29.VIN+ ; also sheet 10
IP30: port D30.VIN+ ; also sheet 10
IP31: port D31.VIN+ ; also sheet 10
ON28: port D28.VOUT+ ; also sheet 10
ON29: port D29.VOUT+ ; also sheet 10
ON30: port D30.VOUT+ ; also sheet 10
ON31: port D31.VOUT+ ; also sheet 10
OP28: port D28.VOUT- ; also sheet 10
OP29: port D29.VOUT- ; also sheet 10
OP30: port D30.VOUT- ; also sheet 10
OP31: port D31.VOUT- ; also sheet 10
V1_8: port D31.VCL D28.VCL D29.VCL D30.VCL ; also sheet 1,2,3,4,5,6,7,8,10
V5: port D28.V5E D29.V5E D30.V5E D31.V5E ; also sheet 1,2,3,4,5,6,7,8,10,12,13
VBIAS [HV]: port D28.VBIAS D29.VBIAS D31.VBIAS D30.VBIAS ; also sheet 1,2,3,4,6,7,8,13
VCOMB: port D28.VCOME D31.VCOME D30.VCOME D29.VCOME ; also sheet 6,7,8,10
VEE: port D28.VEEX D29.VEEX D30.VEEX D31.VEEX ; also sheet 1,2,3,4,6,7,8,12
VTR28: port D28.VTRIM ; also sheet 11
VTR29: port D29.VTRIM ; also sheet 11
VTR30: port D30.VTRIM ; also sheet 11
VTR31: port D31.VTRIM ; also sheet 11

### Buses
OUTBUSB:OP[16..31],ON[16..31]
INBUSB:IP[16..31],IN[16..31]
VTRB:VTR[0..31]

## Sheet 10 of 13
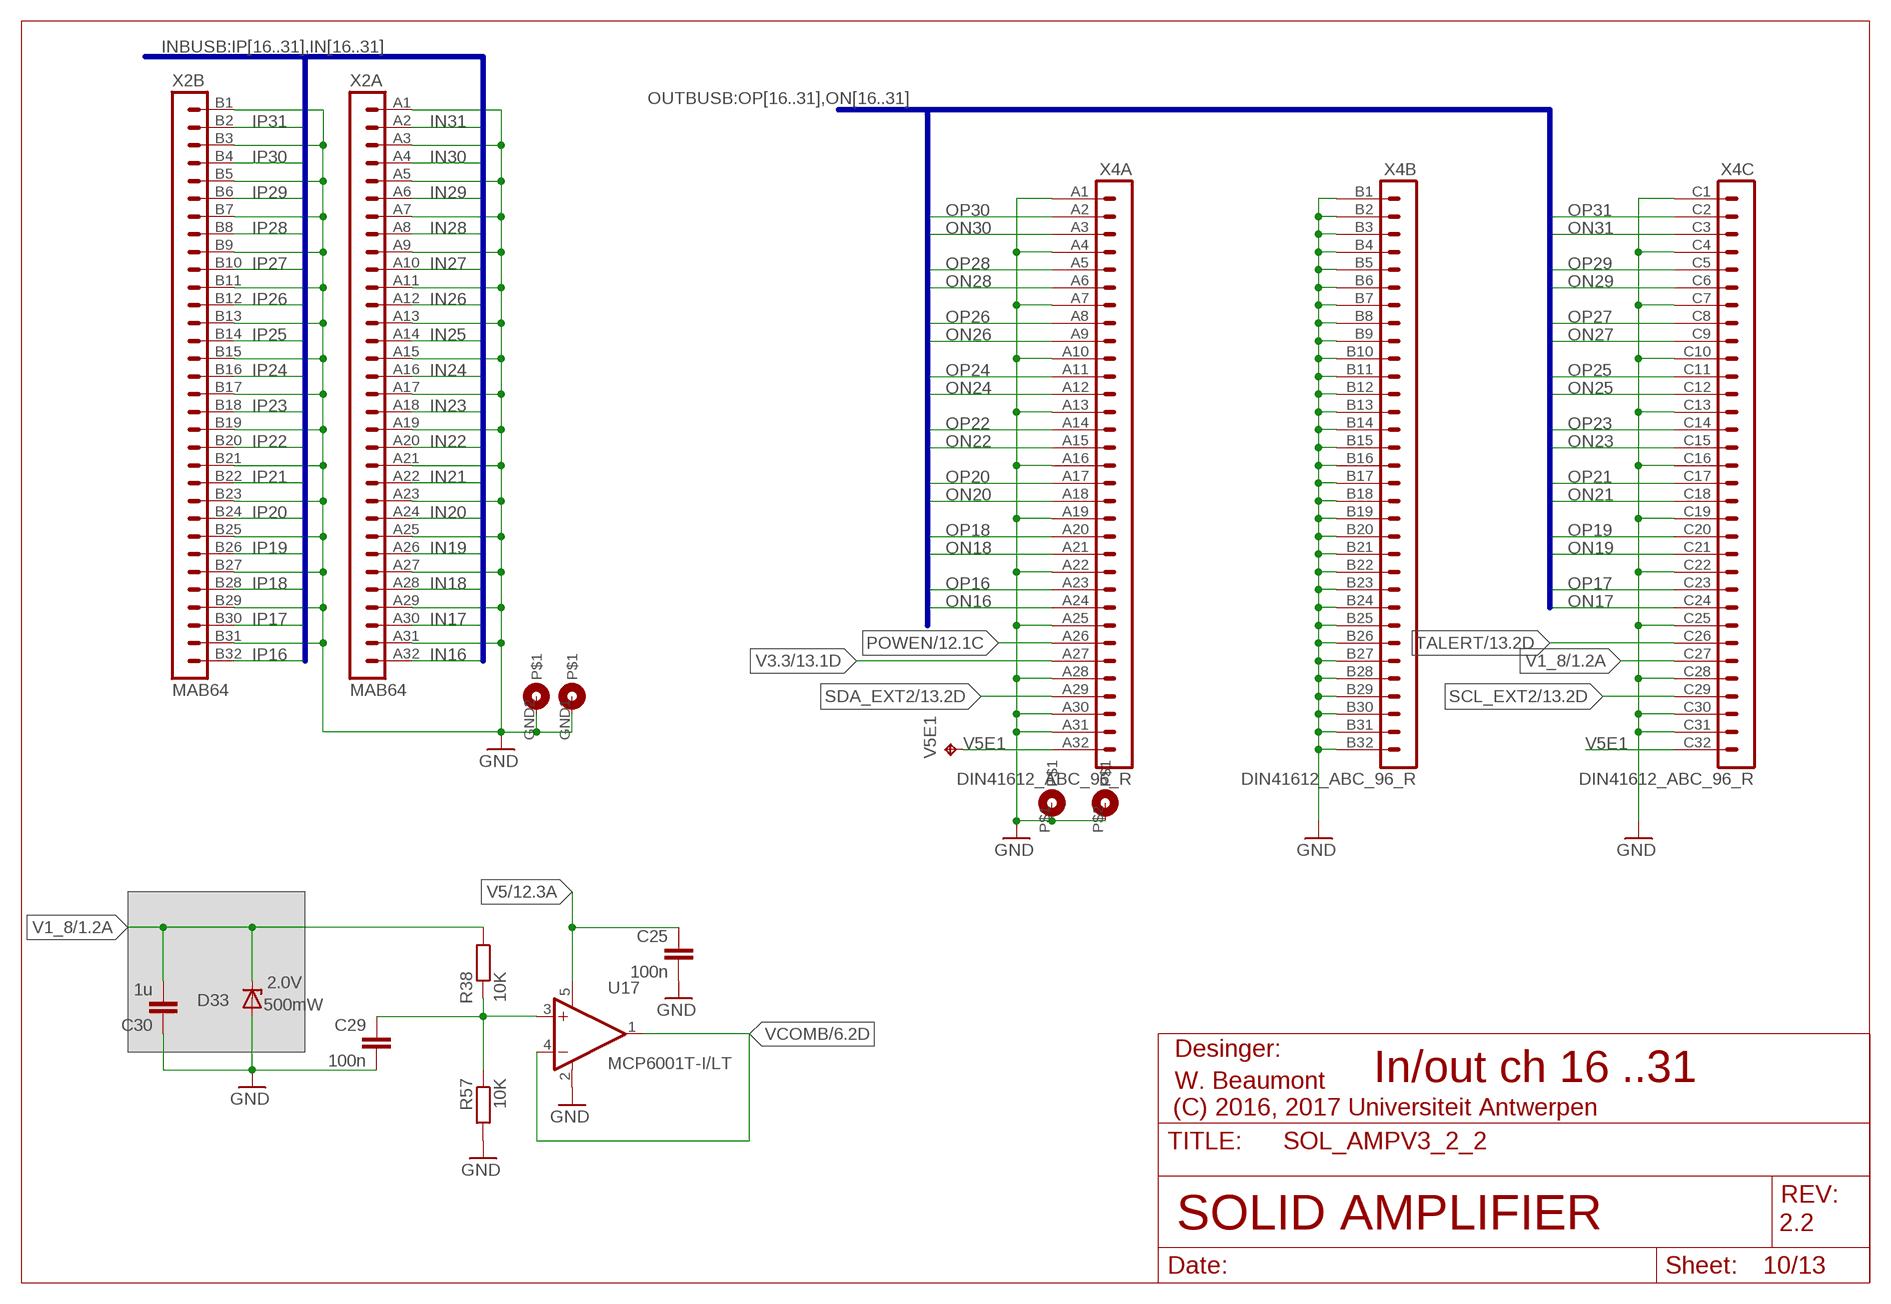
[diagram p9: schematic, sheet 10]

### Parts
C25  100n  C-EUC0402  [C0402]
C29  100n  C-EUC0402  [C0402]
C30  1u  C-EUC0402  [C0402]
D33  2.0V  TFZV  [SOD323R_ROHM]
R38  10K  R-EU_R0402  [R0402]
R57  10K  R-EU_R0402  [R0402]
U17  MCP6001T-I/LT  [SOT65P240X110-5N]
V5E1  UA_TPPAD1-13  [UA_P1-13]
X2  MAB64  [MAB64]
X4  DIN41612_ABC_96_R  [DIN41612_96RC]

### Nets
GND: C25.2 C29.2 C30.1 D33.A R57.2 U17.2(V-) X2.A1 X2.A3 X2.A5 X2.A7 X2.A9 X2.A11 X2.A13 X2.A15 X2.A17 X2.A19 X2.A21 X2.A23 X2.A25 X2.A27 X2.A29 X2.A31 X2.B1 X2.B3 X2.B5 X2.B7 X2.B9 X2.B11 X2.B13 X2.B15 X2.B17 X2.B19 X2.B21 X2.B23 X2.B25 X2.B27 X2.B29 X2.B31 X2.GND1 X2.GND2 X4.A1 X4.A4 X4.A7 X4.A10 X4.A13 X4.A16 X4.A19 X4.A22 X4.A25 X4.A28 X4.A30 X4.A31 X4.B1 X4.B2 X4.B3 X4.B4 X4.B5 X4.B6 X4.B7 X4.B8 X4.B9 X4.B10 X4.B11 X4.B12 X4.B13 X4.B14 X4.B15 X4.B16 X4.B17 X4.B18 X4.B19 X4.B20 X4.B21 X4.B22 X4.B23 X4.B24 X4.B25 X4.B26 X4.B27 X4.B28 X4.B29 X4.B30 X4.B31 X4.B32 X4.C1 X4.C4 X4.C7 X4.C10 X4.C13 X4.C16 X4.C19 X4.C22 X4.C25 X4.C28 X4.C30 X4.C31 X4.P$1 X4.P$2 ; also sheet 1,2,3,4,5,6,7,8,9,11,12,13
IN16: X2.A32 ; also sheet 6
IN17: X2.A30 ; also sheet 6
IN18: X2.A28 ; also sheet 6
IN19: X2.A26 ; also sheet 6
IN20: X2.A24 ; also sheet 7
IN21: X2.A22 ; also sheet 7
IN22: X2.A20 ; also sheet 7
IN23: X2.A18 ; also sheet 7
IN24: X2.A16 ; also sheet 8
IN25: X2.A14 ; also sheet 8
IN26: X2.A12 ; also sheet 8
IN27: X2.A10 ; also sheet 8
IN28: X2.A8 ; also sheet 9
IN29: X2.A6 ; also sheet 9
IN30: X2.A4 ; also sheet 9
IN31: X2.A2 ; also sheet 9
IP16: X2.B32 ; also sheet 6
IP17: X2.B30 ; also sheet 6
IP18: X2.B28 ; also sheet 6
IP19: X2.B26 ; also sheet 6
IP20: X2.B24 ; also sheet 7
IP21: X2.B22 ; also sheet 7
IP22: X2.B20 ; also sheet 7
IP23: X2.B18 ; also sheet 7
IP24: X2.B16 ; also sheet 8
IP25: X2.B14 ; also sheet 8
IP26: X2.B12 ; also sheet 8
IP27: X2.B10 ; also sheet 8
IP28: X2.B8 ; also sheet 9
IP29: X2.B6 ; also sheet 9
IP30: X2.B4 ; also sheet 9
IP31: X2.B2 ; also sheet 9
N$2: C29.1 R38.2 R57.1 U17.3(+IN)
ON16: X4.A24 ; also sheet 6
ON17: X4.C24 ; also sheet 6
ON18: X4.A21 ; also sheet 6
ON19: X4.C21 ; also sheet 6
ON20: X4.A18 ; also sheet 7
ON21: X4.C18 ; also sheet 7
ON22: X4.A15 ; also sheet 7
ON23: X4.C15 ; also sheet 7
ON24: X4.A12 ; also sheet 8
ON25: X4.C12 ; also sheet 8
ON26: X4.A9 ; also sheet 8
ON27: X4.C9 ; also sheet 8
ON28: X4.A6 ; also sheet 9
ON29: X4.C6 ; also sheet 9
ON30: X4.A3 ; also sheet 9
ON31: X4.C3 ; also sheet 9
OP16: X4.A23 ; also sheet 6
OP17: X4.C23 ; also sheet 6
OP18: X4.A20 ; also sheet 6
OP19: X4.C20 ; also sheet 6
OP20: X4.A17 ; also sheet 7
OP21: X4.C17 ; also sheet 7
OP22: X4.A14 ; also sheet 7
OP23: X4.C14 ; also sheet 7
OP24: X4.A11 ; also sheet 8
OP25: X4.C11 ; also sheet 8
OP26: X4.A8 ; also sheet 8
OP27: X4.C8 ; also sheet 8
OP28: X4.A5 ; also sheet 9
OP29: X4.C5 ; also sheet 9
OP30: X4.A2 ; also sheet 9
OP31: X4.C2 ; also sheet 9
POWEN: X4.A26 ; also sheet 12
SCL_EXT2: X4.C29 ; also sheet 13
SDA_EXT2: X4.A29 ; also sheet 13
TALERT: X4.C26 ; also sheet 13
V1_8: C30.2 D33.C R38.1 X4.C27 ; also sheet 1,2,3,4,5,6,7,8,9
V3.3: X4.A27 ; also sheet 5,13
V5: C25.1 U17.5(V+) ; also sheet 1,2,3,4,5,6,7,8,9,12,13
V5E1: V5E1.TP X4.A32 X4.C32
VCOMB: U17.1(OUT) U17.4(-IN) ; also sheet 6,7,8,9

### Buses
INBUSB:IP[16..31],IN[16..31]
OUTBUSB:OP[16..31],ON[16..31]

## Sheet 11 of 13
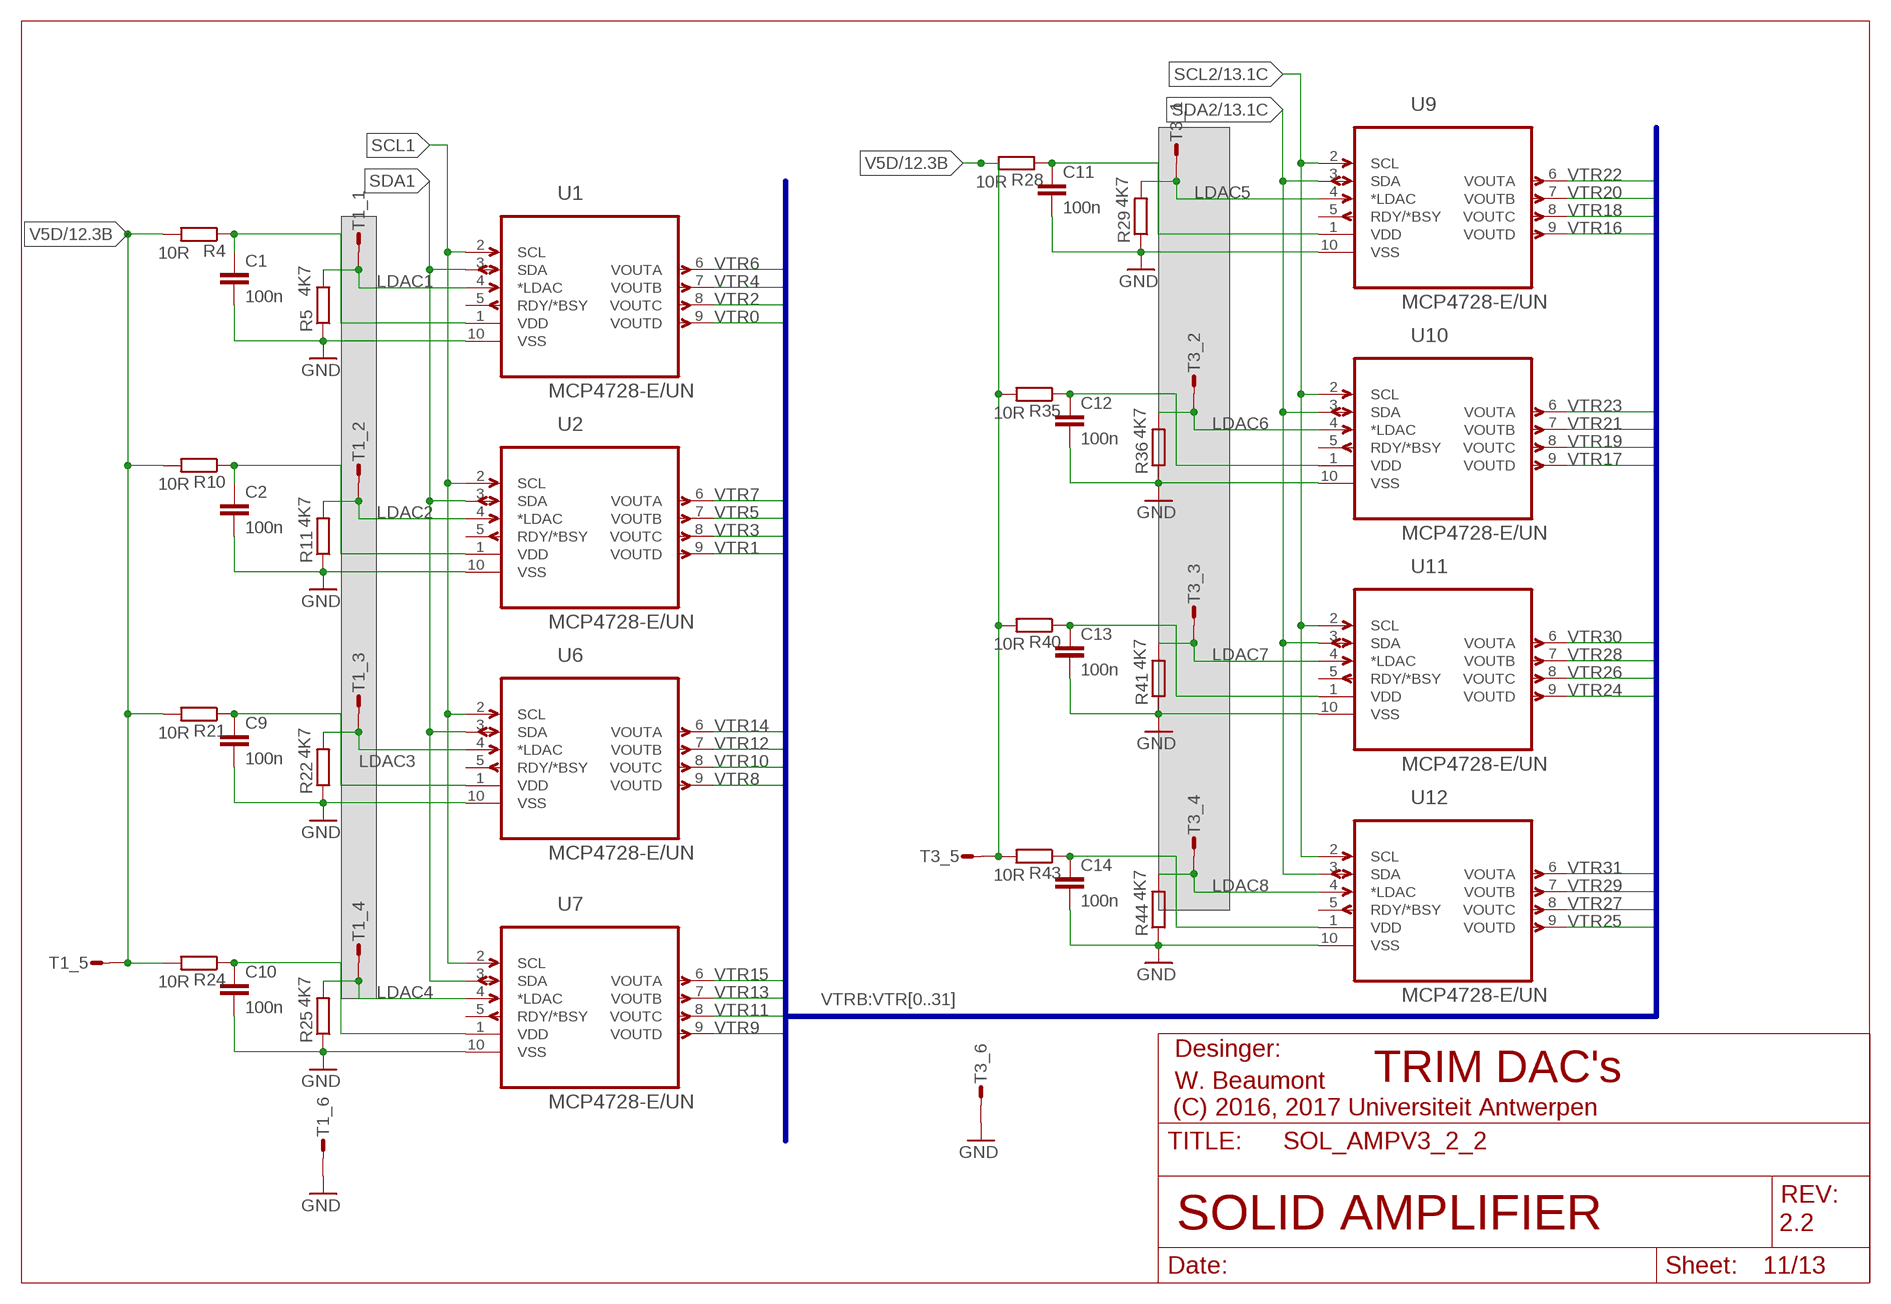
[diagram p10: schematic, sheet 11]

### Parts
C1  100n  C-EUC0402  [C0402]
C2  100n  C-EUC0402  [C0402]
C9  100n  C-EUC0402  [C0402]
C10  100n  C-EUC0402  [C0402]
C11  100n  C-EUC0402  [C0402]
C12  100n  C-EUC0402  [C0402]
C13  100n  C-EUC0402  [C0402]
C14  100n  C-EUC0402  [C0402]
R4  10R  R-EU_R0402  [R0402]
R5  4K7  R-EU_R0402  [R0402]
R10  10R  R-EU_R0402  [R0402]
R11  4K7  R-EU_R0402  [R0402]
R21  10R  R-EU_R0402  [R0402]
R22  4K7  R-EU_R0402  [R0402]
R24  10R  R-EU_R0402  [R0402]
R25  4K7  R-EU_R0402  [R0402]
R28  10R  R-EU_R0402  [R0402]
R29  4K7  R-EU_R0402  [R0402]
R35  10R  R-EU_R0402  [R0402]
R36  4K7  R-EU_R0402  [R0402]
R40  10R  R-EU_R0402  [R0402]
R41  4K7  R-EU_R0402  [R0402]
R43  10R  R-EU_R0402  [R0402]
R44  4K7  R-EU_R0402  [R0402]
T1  NC  UATP2X3  [UATP2X3]
T3  NC  UATP2X3  [UATP2X3]
U1  MCP4728-E/UN  [SOP50P490X110-10N]
U2  MCP4728-E/UN  [SOP50P490X110-10N]
U6  MCP4728-E/UN  [SOP50P490X110-10N]
U7  MCP4728-E/UN  [SOP50P490X110-10N]
U9  MCP4728-E/UN  [SOP50P490X110-10N]
U10  MCP4728-E/UN  [SOP50P490X110-10N]
U11  MCP4728-E/UN  [SOP50P490X110-10N]
U12  MCP4728-E/UN  [SOP50P490X110-10N]

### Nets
GND: C1.2 C2.2 C9.2 C10.2 C11.2 C12.2 C13.2 C14.2 R5.1 R11.1 R22.1 R25.1 R29.1 R36.1 R41.1 R44.1 T1.6 T3.6 U1.10(VSS) U2.10(VSS) U6.10(VSS) U7.10(VSS) U9.10(VSS) U10.10(VSS) U11.10(VSS) U12.10(VSS) ; also sheet 1,2,3,4,5,6,7,8,9,10,12,13
LDAC1: R5.2 T1.1 U1.4(*LDAC)
LDAC2: R11.2 T1.2 U2.4(*LDAC)
LDAC3: R22.2 T1.3 U6.4(*LDAC)
LDAC4: R25.2 T1.4 U7.4(*LDAC)
LDAC5: R29.2 T3.1 U9.4(*LDAC)
LDAC6: R36.2 T3.2 U10.4(*LDAC)
LDAC7: R41.2 T3.3 U11.4(*LDAC)
LDAC8: R44.2 T3.4 U12.4(*LDAC)
N$1: C1.1 R4.1 U1.1(VDD)
N$6: C2.1 R10.1 U2.1(VDD)
N$8: C9.1 R21.1 U6.1(VDD)
N$11: C10.1 R24.1 U7.1(VDD)
N$12: C11.1 R28.1 U9.1(VDD)
N$14: C12.1 R35.1 U10.1(VDD)
N$15: C13.1 R40.1 U11.1(VDD)
N$16: C14.1 R43.1 U12.1(VDD)
SCL1: U1.2(SCL) U2.2(SCL) U6.2(SCL) U7.2(SCL) ; also sheet 13
SCL2: U9.2(SCL) U10.2(SCL) U11.2(SCL) U12.2(SCL) ; also sheet 13
SDA1: U1.3(SDA) U2.3(SDA) U6.3(SDA) U7.3(SDA) ; also sheet 13
SDA2: U9.3(SDA) U10.3(SDA) U11.3(SDA) U12.3(SDA) ; also sheet 13
V5D: R4.2 R10.2 R21.2 R24.2 R28.2 R35.2 R40.2 R43.2 T1.5 T3.5 ; also sheet 12,13
VTR0: U1.9(VOUTD) ; also sheet 1
VTR1: U2.9(VOUTD) ; also sheet 1
VTR2: U1.8(VOUTC) ; also sheet 1
VTR3: U2.8(VOUTC) ; also sheet 1
VTR4: U1.7(VOUTB) ; also sheet 2
VTR5: U2.7(VOUTB) ; also sheet 2
VTR6: U1.6(VOUTA) ; also sheet 2
VTR7: U2.6(VOUTA) ; also sheet 2
VTR8: U6.9(VOUTD) ; also sheet 3
VTR9: U7.9(VOUTD) ; also sheet 3
VTR10: U6.8(VOUTC) ; also sheet 3
VTR11: U7.8(VOUTC) ; also sheet 3
VTR12: U6.7(VOUTB) ; also sheet 4
VTR13: U7.7(VOUTB) ; also sheet 4
VTR14: U6.6(VOUTA) ; also sheet 4
VTR15: U7.6(VOUTA) ; also sheet 4
VTR16: U9.9(VOUTD) ; also sheet 6
VTR17: U10.9(VOUTD) ; also sheet 6
VTR18: U9.8(VOUTC) ; also sheet 6
VTR19: U10.8(VOUTC) ; also sheet 6
VTR20: U9.7(VOUTB) ; also sheet 7
VTR21: U10.7(VOUTB) ; also sheet 7
VTR22: U9.6(VOUTA) ; also sheet 7
VTR23: U10.6(VOUTA) ; also sheet 7
VTR24: U11.9(VOUTD) ; also sheet 8
VTR25: U12.9(VOUTD) ; also sheet 8
VTR26: U11.8(VOUTC) ; also sheet 8
VTR27: U12.8(VOUTC) ; also sheet 8
VTR28: U11.7(VOUTB) ; also sheet 9
VTR29: U12.7(VOUTB) ; also sheet 9
VTR30: U11.6(VOUTA) ; also sheet 9
VTR31: U12.6(VOUTA) ; also sheet 9
Unconnected: U1.5(RDY/*BSY) U2.5(RDY/*BSY) U6.5(RDY/*BSY) U7.5(RDY/*BSY) U9.5(RDY/*BSY) U10.5(RDY/*BSY) U11.5(RDY/*BSY) U12.5(RDY/*BSY)

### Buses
VTRB:VTR[0..31]

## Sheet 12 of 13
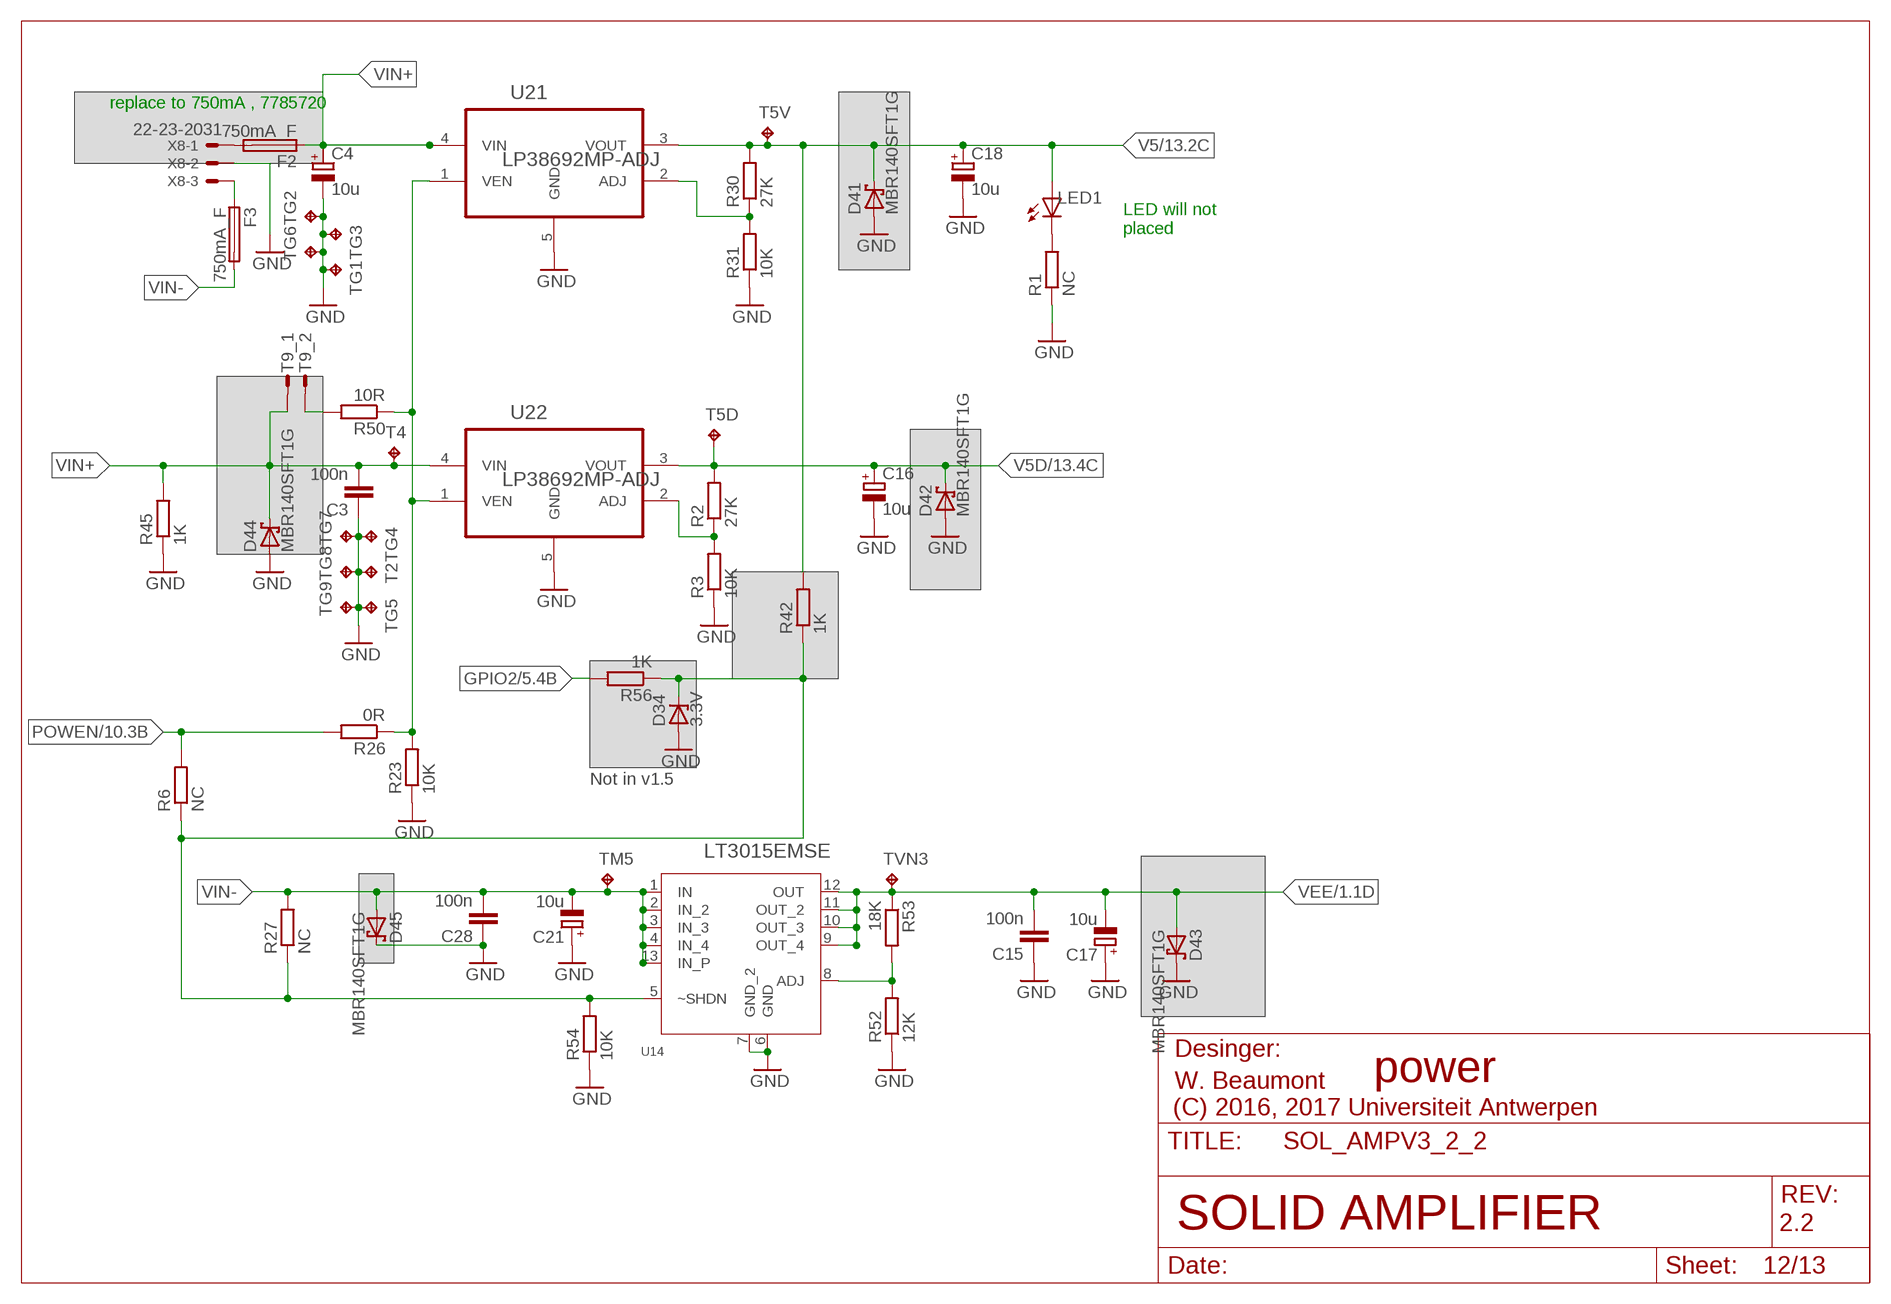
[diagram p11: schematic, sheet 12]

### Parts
C3  100n  C-EUC0402  [C0402]
C4  10u  CPOL-EUSMCA  [SMC_A]
C15  100n  C-EUC0402  [C0402]
C16  10u  CPOL-EUSMCA  [SMC_A]
C17  10u  CPOL-EUSMCA  [SMC_A]
C18  10u  CPOL-EUSMCA  [SMC_A]
C21  10u  CPOL-EUSMCA  [SMC_A]
C28  100n  C-EUC0402  [C0402]
D34  3.3V  UDZVF  [SOD323F_ROHM]
D41  MBR140SFT1G  [SOD123FL]
D42  MBR140SFT1G  [SOD123FL]
D43  MBR140SFT1G  [SOD123FL]
D44  MBR140SFT1G  [SOD123FL]
D45  MBR140SFT1G  [SOD123FL]
F2  750mA_F  FUSEFUSE750MA  [FUSE1206]
F3  750mA_F  FUSEFUSE750MA  [FUSE1206]
LED1  NC  LEDCHIP-LED0805  [CHIP-LED0805]
R1  NC  R-EU_R0402  [R0402]
R2  27K  R-EU_R0402  [R0402]
R3  10K  R-EU_R0402  [R0402]
R6  NC  R-EU_R0402  [R0402]
R23  10K  R-EU_R0402  [R0402]
R26  0R  R-EU_R0402  [R0402]
R27  NC  R-EU_R0402  [R0402]
R30  27K  R-EU_R0402  [R0402]
R31  10K  R-EU_R0402  [R0402]
R42  1K  R-EU_R0402  [R0402]
R45  1K  R-EU_R0805  [R0805]
R50  10R  R-EU_R0402  [R0402]
R52  12K  R-EU_R0402  [R0402]
R53  18K  R-EU_R0402  [R0402]
R54  10K  R-EU_R0402  [R0402]
R56  1K  R-EU_R0402  [R0402]
T2  UA_TPPAD1-13  [UA_P1-13]
T4  UA_TPPAD1-13  [UA_P1-13]
T5D  UA_TPPAD1-13  [UA_P1-13]
T5V  UA_TPPAD1-13  [UA_P1-13]
T9  NC  UATP1X2  [UATP1X2]
TG1  UA_TPPAD1-13  [UA_P1-13]
TG2  UA_TPPAD1-13  [UA_P1-13]
TG3  UA_TPPAD1-13  [UA_P1-13]
TG4  UA_TPPAD1-13  [UA_P1-13]
TG5  UA_TPPAD1-13  [UA_P1-13]
TG6  UA_TPPAD1-13  [UA_P1-13]
TG7  UA_TPPAD1-13  [UA_P1-13]
TG8  UA_TPPAD1-13  [UA_P1-13]
TG9  UA_TPPAD1-13  [UA_P1-13]
TM5  UA_TPPAD1-13  [UA_P1-13]
TVN3  UA_TPPAD1-13  [UA_P1-13]
U14  LT3015EMSE  LT3015EMSEM  [SOP65P490X110H-13N]
U21  LP38692MP-ADJ  [SOT150P696X180-5N]
U22  LP38692MP-ADJ  [SOT150P696X180-5N]
X8  22-23-2031  [22-23-2031]

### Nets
GND: C3.1 C4.- C15.1 C16.- C17.+ C18.- C21.+ C28.1 D34.A D41.A D42.A D43.C D44.A D45.C R1.1 R3.1 R23.1 R31.1 R45.1 R52.1 R54.1 T2.TP TG1.TP TG2.TP TG3.TP TG4.TP TG5.TP TG6.TP TG7.TP TG8.TP TG9.TP U14.6(GND) U14.7(GND_2) U21.5(GND) U22.5(GND) X8.2 ; also sheet 1,2,3,4,5,6,7,8,9,10,11,13
GPIO2: R56.2 ; also sheet 5
N$3: LED1.C R1.2
N$5: R52.2 R53.2 U14.8(ADJ)
N$20: R30.1 R31.2 U21.2(ADJ)
N$21: F3.1 X8.3
N$22: R2.1 R3.2 U22.2(ADJ)
N$25: F2.2 X8.1
N$27: R50.2 T9.2
POWEN: R6.2 R26.2 ; also sheet 10
POWENP: R23.2 R26.1 R50.1 U21.1(VEN) U22.1(VEN)
V5: C18.+ D41.C LED1.A R30.2 R42.2 T5V.TP U21.3(VOUT) ; also sheet 1,2,3,4,5,6,7,8,9,10,13
V5D: C16.+ D42.C R2.2 T5D.TP U22.3(VOUT) ; also sheet 11,13
VEE: C15.2 C17.- D43.A R53.1 TVN3.TP U14.9(OUT_4) U14.10(OUT_3) U14.11(OUT_2) U14.12(OUT) ; also sheet 1,2,3,4,6,7,8,9
VIN+: C3.2 C4.+ D44.C F2.1 R45.2 T4.TP T9.1 U21.4(VIN) U22.4(VIN)
VIN-: C21.- C28.2 D45.A F3.2 R27.2 TM5.TP U14.1(IN) U14.2(IN_2) U14.3(IN_3) U14.4(IN_4) U14.13(IN_P)
VN3EN: D34.C R6.1 R27.1 R42.1 R54.2 R56.1 U14.5(~SHDN)

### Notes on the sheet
- replace to 750mA , 7785720
- LED will not
  placed
- Not in v1.5

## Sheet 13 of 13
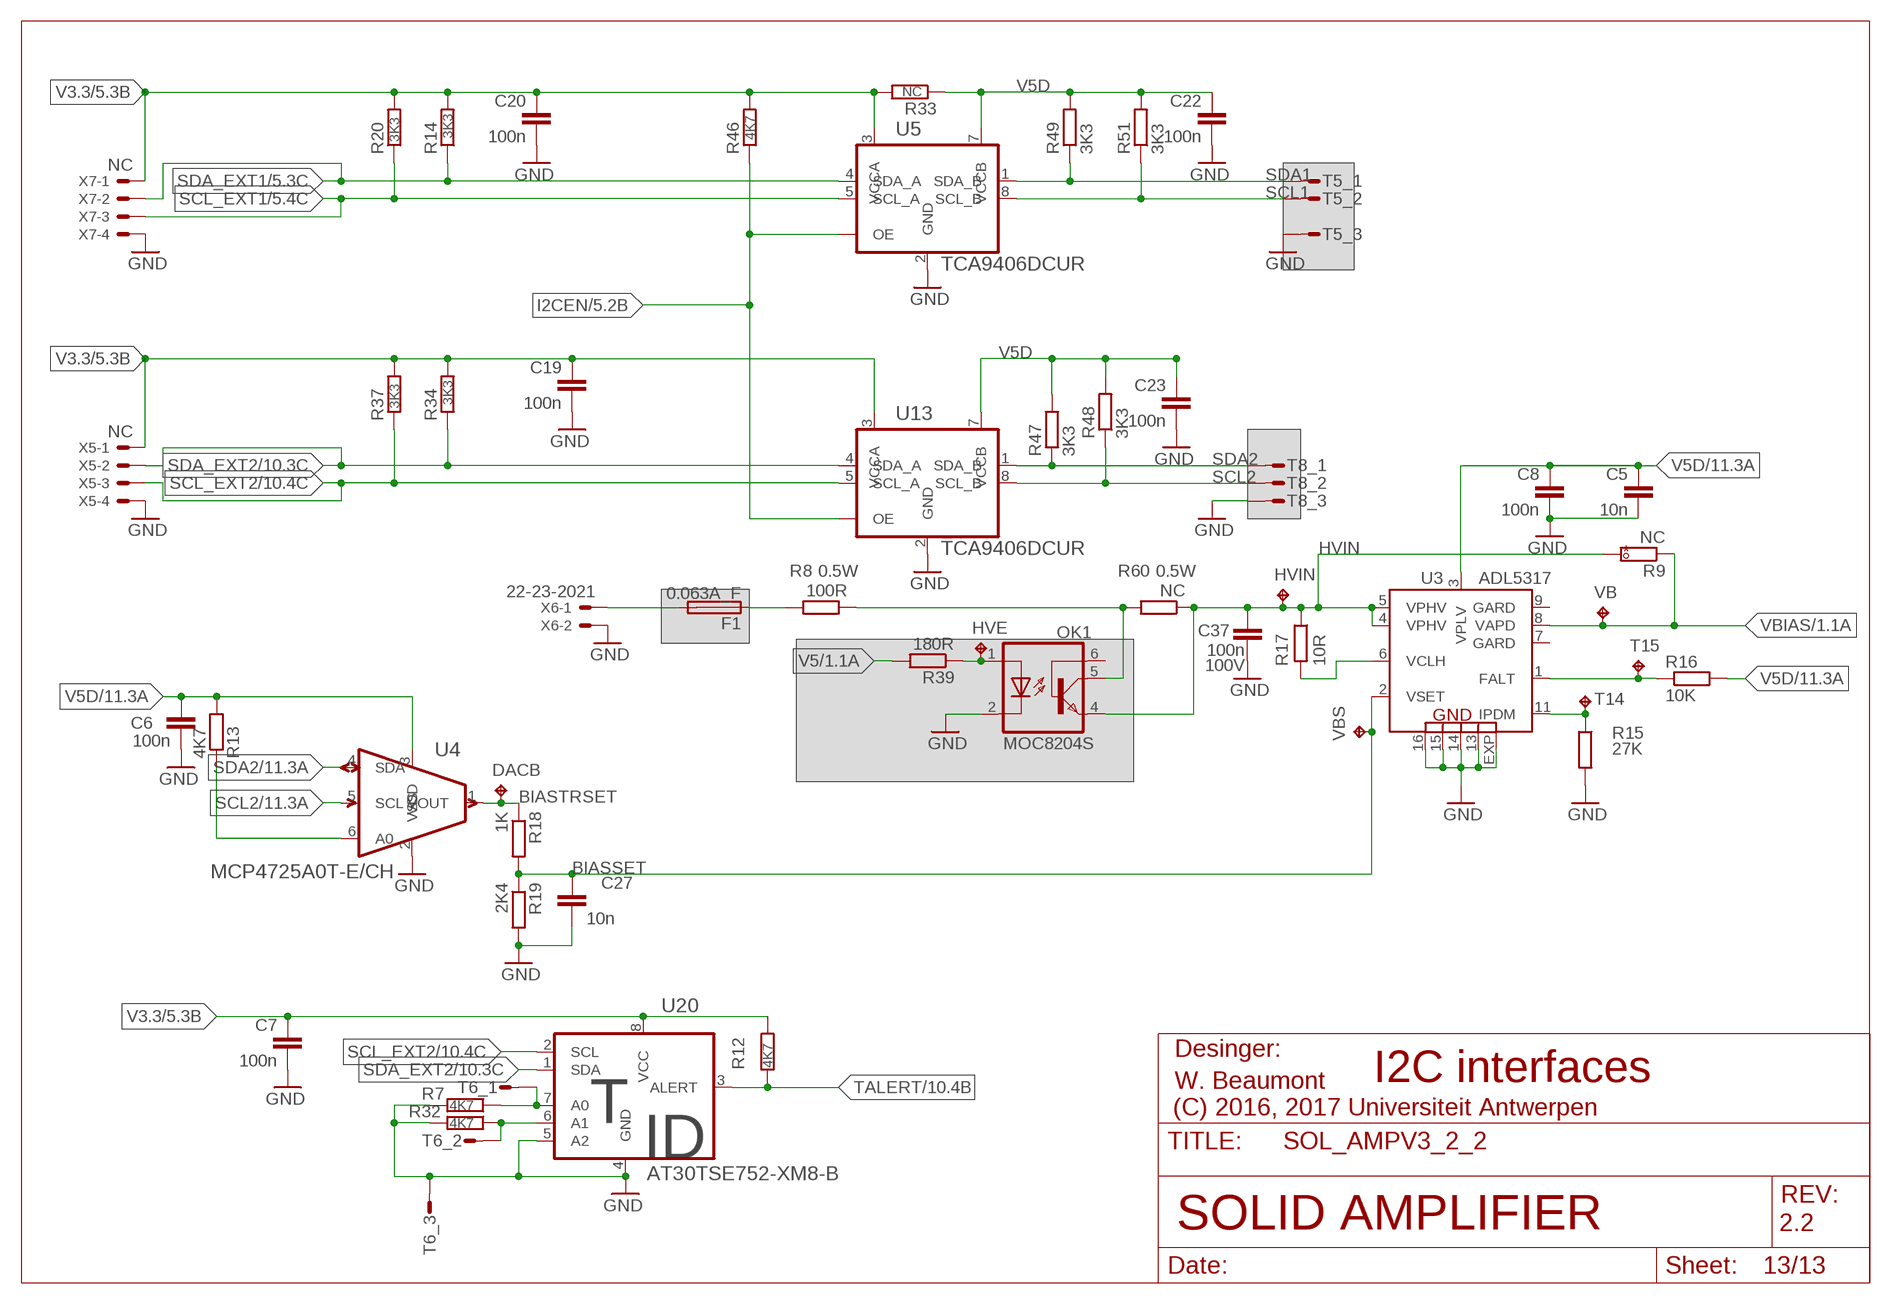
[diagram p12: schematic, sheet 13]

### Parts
C5  10n  C-EUC0402  [C0402]
C6  100n  C-EUC0402  [C0402]
C7  100n  C-EUC0402  [C0402]
C8  100n  C-EUC0402  [C0402]
C19  100n  C-EUC0402  [C0402]
C20  100n  C-EUC0402  [C0402]
C22  100n  C-EUC0402  [C0402]
C23  100n  C-EUC0402  [C0402]
C27  10n  C-EUC0402  [C0402]
C37  100n  C-EUC0603  [C0603]
DACB  UA_TPPAD1-13  [UA_P1-13]
F1  0.063A_F  FUSEOMF62MAOMF  [FUSE7_4X3_1]
HVE  UA_TPPAD1-13  [UA_P1-13]
HVIN  UA_TPPAD1-13  [UA_P1-13]
OK1  MOC8204S  [DIL6-SMD]
R7  4K7  R-EU_R0402  [R0402]
R8  100R  R-EU_M1206  [M1206]
R9  NC  R_HAND  [R0805H]
R12  4K7  R-EU_R0402  [R0402]
R13  4K7  R-EU_R0402  [R0402]
R14  3K3  R-EU_R0402  [R0402]
R15  27K  R-EU_R0402  [R0402]
R16  10K  R-EU_R0402  [R0402]
R17  10R  R-EU_R0805  [R0805]
R18  1K  R-EU_R0402  [R0402]
R19  2K4  R-EU_R0402  [R0402]
R20  3K3  R-EU_R0402  [R0402]
R32  4K7  R-EU_R0402  [R0402]
R33  NC  R-EU_R0402  [R0402]
R34  3K3  R-EU_R0402  [R0402]
R37  3K3  R-EU_R0402  [R0402]
R39  180R  R-EU_R0805  [R0805]
R46  4K7  R-EU_R0402  [R0402]
R47  3K3  R-EU_R0402  [R0402]
R48  3K3  R-EU_R0402  [R0402]
R49  3K3  R-EU_R0402  [R0402]
R51  3K3  R-EU_R0402  [R0402]
R60  NC  R-EU_M1206  [M1206]
T5  UATP1X3  [UATP1X3]
T6  UATP1X3  [UATP1X3]
T8  UATP1X3  [UATP1X3]
T14  UA_TPPAD1-13  [UA_P1-13]
T15  UA_TPPAD1-13  [UA_P1-13]
U3  ADL5317  ADL5317_  [LFCSP_LQ-16]
U4  MCP4725A0T-E/CH  [SOT95P270X145-6N]
U5  TCA9406DCUR  [SOP50P310X90-8N]
U13  TCA9406DCUR  [SOP50P310X90-8N]
U20  AT30TSE752-XM8-B  [SOP65P490X110-8N]
VB  UA_TPPAD1-13  [UA_P1-13]
VBS  UA_TPPAD1-13  [UA_P1-13]
X5  NC  22-23-2041  [22-23-2041]
X6  22-23-2021  [22-23-2021]
X7  NC  22-23-2041  [22-23-2041]

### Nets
BIASSET: C27.1 R18.2 R19.1 U3.2(VSET) VBS.TP
BIASTRSET: DACB.TP R18.1 U4.1(VOUT)
GND: C5.2 C6.2 C7.2 C8.2 C19.2 C20.2 C22.2 C23.2 C27.2 C37.2 OK1.2(C) R7.2 R15.2 R19.2 R32.2 T5.3 T6.3 T8.3 U3.13(GND) U3.14(GND) U3.15(GND) U3.16(GND) U3.EXP(GND) U4.2(VSS) U5.2(GND) U13.2(GND) U20.4(GND) U20.5(A2) X5.4 X6.2 X7.4 ; also sheet 1,2,3,4,5,6,7,8,9,10,11,12
HVCON [HV]: F1.2 X6.1
HVFUSE [HV]: F1.1 R8.2
HVIN [HV]: C37.1 HVIN.TP OK1.4(EMI) R9.2 R17.1 R60.1 U3.4(VPHV) U3.5(VPHV)
HVSW [HV]: OK1.5(COL) R8.1 R60.2
I2CEN: R46.1 U5.6(OE) U13.6(OE) ; also sheet 5
N$4: HVE.TP OK1.1(A) R39.1
N$7: R15.1 T14.TP U3.11(IPDM)
N$9: R17.2 U3.6(VCLH)
N$10: R13.1 U4.6(A0)
N$13: R16.1 T15.TP U3.1(FALT)
SCL1: R51.1 T5.2 U5.8(SCL_B) ; also sheet 11
SCL2: R48.1 T8.2 U4.5(SCL) U13.8(SCL_B) ; also sheet 11
SCL_EXT1: R20.1 U5.5(SCL_A) X7.3 ; also sheet 5
SCL_EXT2: R37.1 U13.5(SCL_A) U20.2(SCL) X5.3 ; also sheet 10
SDA1: R49.1 T5.1 U5.1(SDA_B) ; also sheet 11
SDA2: R47.1 T8.1 U4.4(SDA) U13.1(SDA_B) ; also sheet 11
SDA_EXT1: R14.1 U5.4(SDA_A) X7.2 ; also sheet 5
SDA_EXT2: R34.1 U13.4(SDA_A) U20.1(SDA) X5.2 ; also sheet 10
TALERT: R12.2 U20.3(ALERT) ; also sheet 10
TIDA0: R7.1 T6.1 U20.7(A0)
TIDA1: R32.1 T6.2 U20.6(A1)
V3.3: C7.1 C19.1 C20.1 R12.1 R14.2 R20.2 R33.2 R34.2 R37.2 R46.2 U5.3(VCCA) U13.3(VCCA) U20.8(VCC) X5.1 X7.1 ; also sheet 5,10
V5: R39.2 ; also sheet 1,2,3,4,5,6,7,8,9,10,12
V5D: C5.1 C6.1 C8.1 C22.1 C23.1 R13.2 R16.2 R33.1 R47.2 R48.2 R49.2 R51.2 U3.3(VPLV) U4.3(VDD) U5.7(VCCB) U13.7(VCCB) ; also sheet 11,12
VBIAS [HV]: R9.1 U3.8(VAPD) VB.TP ; also sheet 1,2,3,4,6,7,8,9
Unconnected: OK1.6(BAS) U3.7(GARD) U3.9(GARD)

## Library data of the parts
C1-C3 C5-C15 C19 C20 C22-C29 = rcl:C-EU: CAPACITOR, European symbol
C4 C16-C18 C21 = rcl:CPOL-EU: POLARIZED CAPACITOR, European symbol
C30 C31 = rcl:C-EU: CAPACITOR, European symbol; MOUSER_OC: 81-GRM155R61A105KE15; MPN: GRM155R61A105KE15D; SUPPLIER: MURATA
C37 = rcl:C-EU: CAPACITOR, European symbol; VOLT: 100V
D32 D33 = UA_v2:TFZV: ROHM zener diodes TFZV series & YFZVFH; IMAX: 400mA; MPN: TFZVTR2.0B; OC_FARNELL: 2580911; POWER: 500mW; SUPPLIER: ROHM
D34 = UA_v2:UDZVF: ROHM zener diodes UDZVF series; IMAX: 50mA; MPN: UDZVFHTE-173.3B; OC_FARNELL: 2528863; POWER: 200mW; SUPPLIER: ROHM
D41-D45 = UA_v2:MBR140SFT1G: Schottky 40 V, 1 A SOD-123FL; ALTMPN: MBR130T1; MPN: MBR140SFT1G; OC_FARNELL: 1431046; SUPPLIER: ON SEMCONDUCTOR
DACB HVE HVIN T2 T5D T5V TG4 TG5 TG7-TG9 TM5 TVN3 VBS = UA_v2:UA_TP: Test pad
F1 = UA_v2:FUSE; MOUSER_OC: 693-3404.0003.11; MPN: 3413.0008.22; RC_OC: 3404.0003.11; SUPPLIER: Schurter; VAC: 125; VDC: 125
F2 F3 = UA_v2:FUSE; MPN: 3413.0114.22; OC_FARNELL: 7785720; SUPPLIER: SCHURTER; VAC: 125; VDC: 125
GPIO2 T4 T14 T15 TG1-TG3 TG6 V5E1 V5E2 VB = UA_v2:UA_TP: Test pad; PARTNO: *
LED1 = led:LED: LED; MPN: HSMG-C170
OK1 = UA_v2:MOC8204: General Purpose 6-Pin Phototransistor Optocouplers Source: http://www.fairchildsemi.com/ds/4N/4N35-M.pdf; MPN: MOC8204SR2M; OC_FARNELL: 2322563; SUPPLIER: FAIRCHILD
R1-R5 R7 R10-R26 R28-R59 = rcl:R-EU_: RESISTOR, European symbol
R6 R27 = rcl:R-EU_: RESISTOR, European symbol; PARTNO: *
R8 R60 = rcl:R-EU_: RESISTOR, European symbol; POWER: 0.5W
R9 = UA_v2:R_HAND; PARTNO: *
T1 T3 = UA_v2:UATP2X3: Holes are smaller for a kind of press fitting. Not intention to have the header placed only temporarily for testing / programming purposes
T5 T6 T8 = UA_v2:UATP1X3: TP group header with smaller holes not intendet for placing a header only for test point
T9 T10 = UA_v2:UATP1X2: TP group header with smaller holes not intendet for placing a header only for test point
U1 U2 U6 U7 U9-U12 = MCP4728:MCP4728-E/UN: IC, DAC, 12BIT, QUAD; MPN: MCP4728-E/UN; OC_FARNELL: 1800217; OC_NEWARK: 08R1808; PACKAGE: MSOP-10; SUPPLIER: MICROCHIP
U3 = ua_cmp:ADL5317: APD voltage regulator; MPN: ADL5317ACPZ; OC_FARNELL: 2462433
U4 = ua_cmp:MCP4725A0T-E/CH: 12-Bit Digital-to-Analog Converter with EEPROM; MPN: MCP4725A0T-E/CH; OC_FARNELL: 1578449; OC_NEWARK: 77M3032; PACKAGE: SOT-23-6; SUPPLIER: Microchip
U5 U13 = TCA9406D:TCA9406DCUR: 2-BIT BIDIRECTIONAL 1MHz, I2C BUS AND SMBUS VOLTAGE-LEVEL TRANSLATOR WITH 8kV HBM ESD,US8-8; MOUSER_OC: 595-TCA9406DCUR; MPN: TCA9406DCUR; OC_FARNELL: 1972385; OC_NEWARK: 86W6769; PACKAGE: US8-8; SUPPLIER: TEXAS INSTRUMENTS
U14 = LT3050:LT3015EMSE: Linear Regulator; MPN: LT3015EMSE; OC_FARNELL: 2068044; PACKAGE: MSOP-12; SUPPLIER: Linear Technology
U17 U19 = MCP6001T:MCP6001T-I/LT: IC OPAMP 1.8V 1MHZ SINGLE; MPN: MCP6001T-I/LT; OC_FARNELL: 8540837; OC_NEWARK: 89K2099; PACKAGE: SC70-5; SUPPLIER: Microchip
U20 = at305sse752:AT30TSE752-XM8-B: SENSOR, TEMP, 9-12BIT, 2KB EEPROM, MSOP-8; MPN: AT30TSE752-XM8-B; OC_FARNELL: 2115206; OC_NEWARK: Unknown; PACKAGE: MSOP-8; SUPPLIER: ATMEL
U21 U22 = UA_v2:LP38692MP-ADJ: Linear Regulator; MPN: LP38692MP-ADJ; OC_FARNELL: 1008058; OC_NEWARK: 41K7473; PACKAGE: SOT-223-5; SUPPLIER: NationalSemiconductor
X1 X2 = SOL_AMPV3specials:MAB64: CONNECTOR DIN 41612 Connector, Type B Series, 64 Plug, 2.54 mm, 2 Row, a + b; MPN: 09 02 164 7921; OC_FARNELL: 1096830; SUPPLIER: HARTING
X3 X4 = SOL_AMPV3specials:DIN41612_ABC_96_R: DIN 41612 Connector, 96 Receptacle, 2.54 mm, 3 Row, a + b + c; MPN: 0973 296 6801; OC_FARNELL: 1096942; SUPPLIER: HARTING
X5 X7 = con-molex:22-23-2041: .100 inch (2.54mm) Center Header - 4 Pin; MPN: 22-23-2041; OC_FARNELL: 1462920; OC_NEWARK: 38C0355; SUPPLIER: MOLEX
X6 = con-molex:22-23-2021: .100 inch (2.54mm) Center Header - 2 Pin; MPN: 22-23-2021; OC_FARNELL: 1462926; OC_NEWARK: 25C3832; SUPPLIER: MOLEX
X8 = con-molex:22-23-2031: .100 inch (2.54mm) Center Header - 3 Pin; MPN: 22-23-2031; OC_FARNELL: 1462950; OC_NEWARK: 30C0862; SUPPLIER: MOLEX

## Module DIFFAMP$B
Ports: VIN+(in) VIN-(in) VTRIM(in) V5E(pwr) GNDE(pwr) VBIAS(in) VOUT+(out) VOUT-(out) VEEX(pwr) VCOME(in) VCL(in)
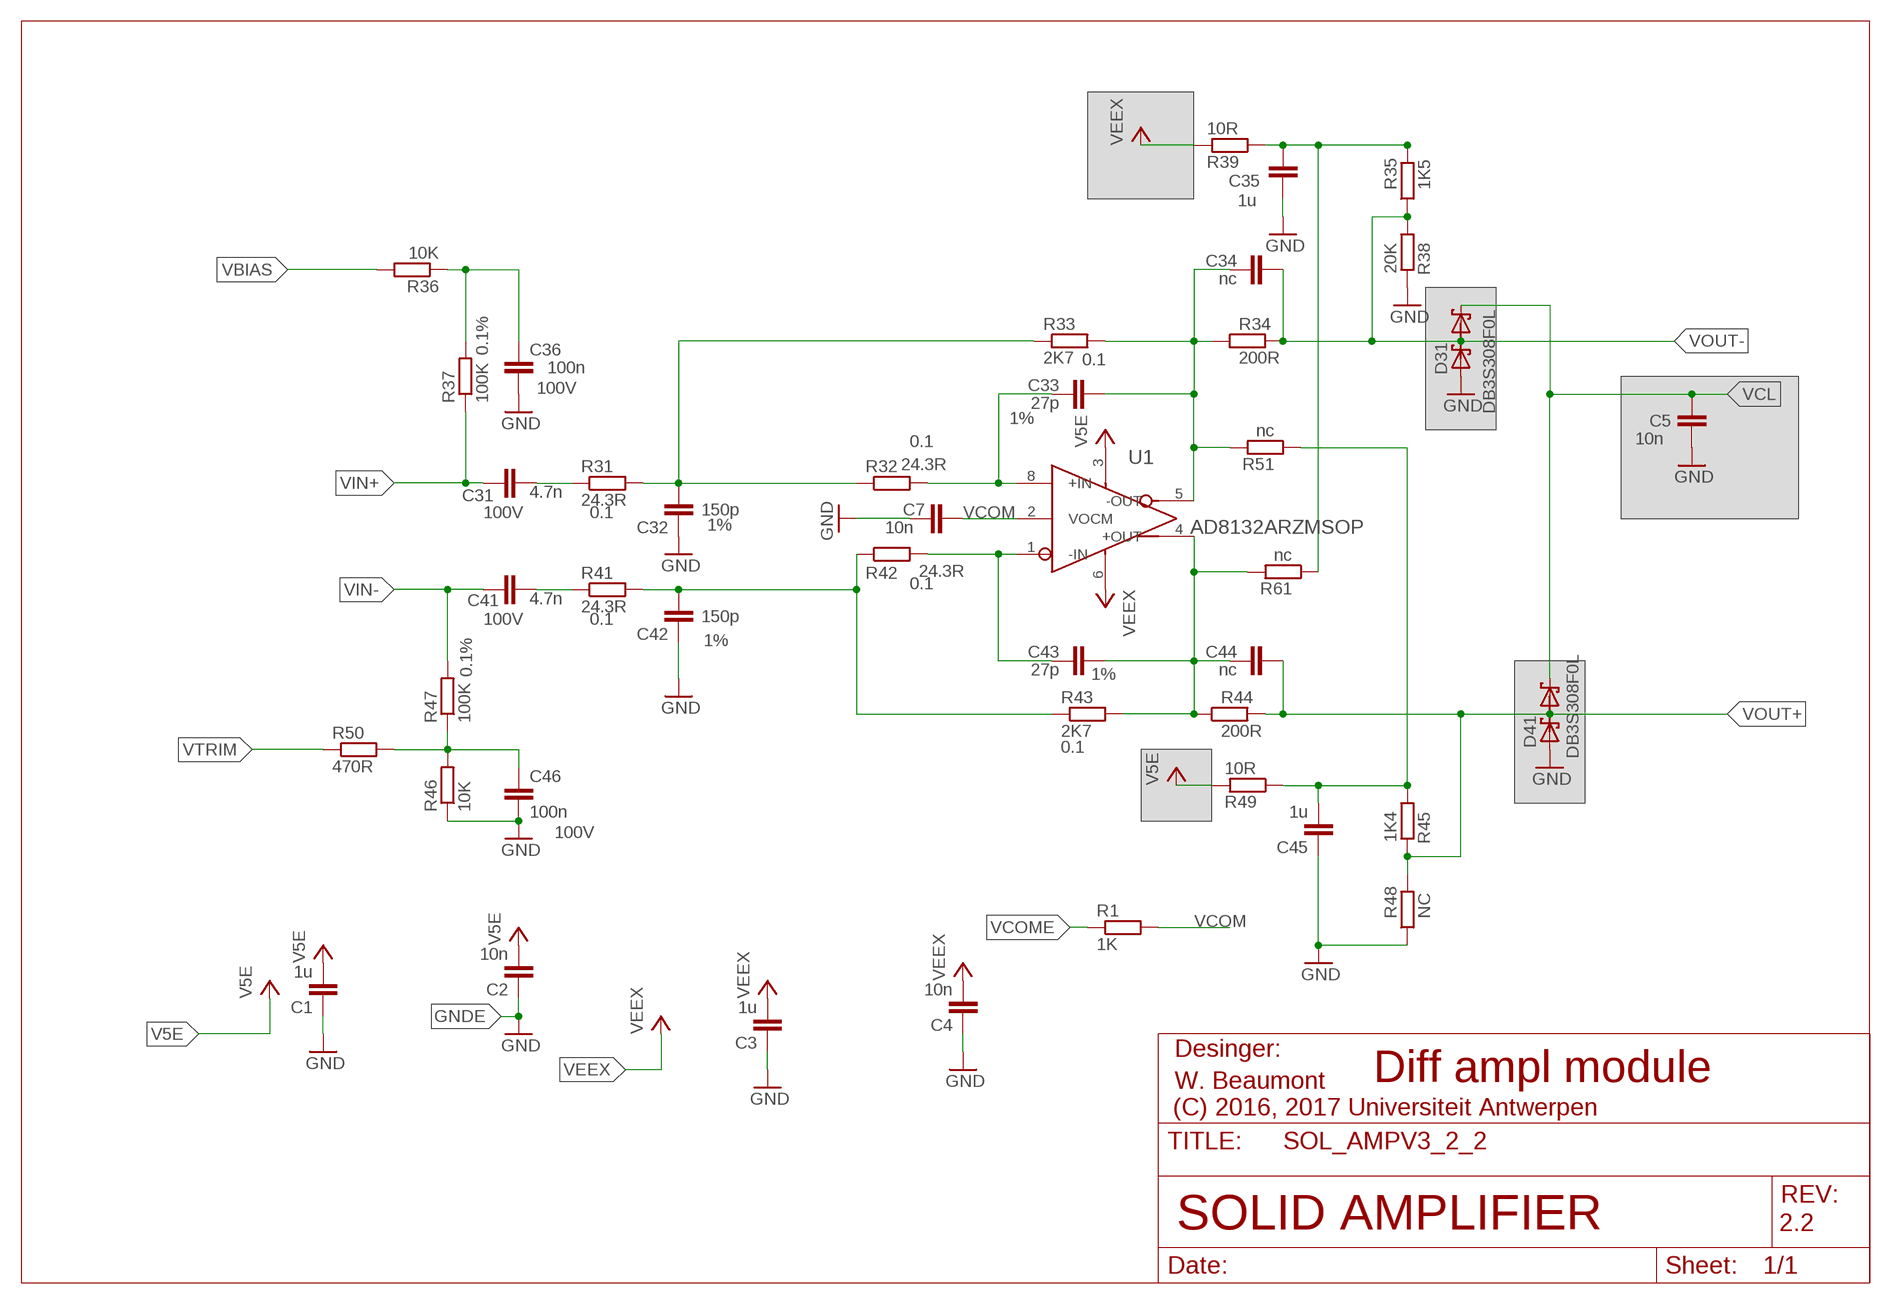
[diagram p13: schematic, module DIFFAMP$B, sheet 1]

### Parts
C1  1u  C-EUC0402  [C0402]
C2  10n  C-EUC0402  [C0402]
C3  1u  C-EUC0402  [C0402]
C4  10n  C-EUC0402  [C0402]
C5  10n  C-EUC0402  [C0402]
C7  10n  C-EUC0402  [C0402]
C31  4.7n  C-EUC0603  [C0603]
C32  150p  C-EUC0402  [C0402]
C33  27p  C-EUC0402  [C0402]
C34  nc  C-EUC0402  [C0402]
C35  1u  C-EUC0402  [C0402]
C36  100n  C-EUC0603  [C0603]
C41  4.7n  C-EUC0603  [C0603]
C42  150p  C-EUC0402  [C0402]
C43  27p  C-EUC0402  [C0402]
C44  nc  C-EUC0402  [C0402]
C45  1u  C-EUC0402  [C0402]
C46  100n  C-EUC0603  [C0603]
D31  DB3S308F0L  DB3S308F  [SOT490]
D41  DB3S308F0L  DB3S308F  [SOT490]
R1  1K  R-EU_R0402  [R0402]
R31  24.3R  R-EU_R0603  [R0603]
R32  24.3R  R-EU_R0603  [R0603]
R33  2K7  R-EU_R0603  [R0603]
R34  200R  R-EU_R0402  [R0402]
R35  1K5  R-EU_R0402  [R0402]
R36  10K  R-EU_R0402  [R0402]
R37  100K  R-EU_R0603  [R0603]
R38  20K  R-EU_R0402  [R0402]
R39  10R  R-EU_R0402  [R0402]
R41  24.3R  R-EU_R0603  [R0603]
R42  24.3R  R-EU_R0603  [R0603]
R43  2K7  R-EU_R0603  [R0603]
R44  200R  R-EU_R0402  [R0402]
R45  1K4  R-EU_R0402  [R0402]
R46  10K  R-EU_R0402  [R0402]
R47  100K  R-EU_R0603  [R0603]
R48  NC  R-EU_R0402  [R0402]
R49  10R  R-EU_R0402  [R0402]
R50  470R  R-EU_R0402  [R0402]
R51  nc  R-EU_R0402  [R0402]
R61  nc  R-EU_R0402  [R0402]
U1  AD8132ARZMSOP  [SOP65P490X110-8N]

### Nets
AMP+: C43.2 C44.1 R43.2 R44.1 R61.2 U1.4(+OUT)
AMP-: C33.2 C34.1 R33.2 R34.1 R51.2 U1.5(-OUT)
FB+: C32.2 R31.2 R32.1 R33.1
FB-: C42.2 R41.2 R42.1 R43.1
GNDE: C1.1 C2.1 C3.1 C4.1 C5.1 C7.2 C32.1 C35.1 C36.2 C42.1 C45.1 C46.2 D31.1 D41.1 R38.2 R46.1 R48.1 ; supply symbol labelled GND
N$1: C45.2 R45.1 R49.1 R51.1
N$4: C43.1 R42.2 U1.1(-IN)
N$5: C33.1 R32.2 U1.8(+IN)
N$7: C35.2 R35.2 R39.1 R61.1
N$10: C41.1 R41.1
R31: C31.1 R31.1
V5E: C1.2 C2.2 R49.2 U1.3(V+)
VB+ [HV]: C36.1 R36.1 R37.2
VB-: C46.1 R46.2 R47.1 R50.2
VBIAS [HV]: R36.2
VCL: C5.2 D31.2 D41.2
VCOM: C7.1 R1.2 U1.2(VOCM)
VCOME: R1.1
VEEX: C3.2 C4.2 R39.2 U1.6(V-)
VIN+ [HV]: C31.2 R37.1
VIN-: C41.2 R47.2
VOUT+: C44.2 D41.3 R44.2 R45.2 R48.2
VOUT-: C34.2 D31.3 R34.2 R35.1 R38.1
VTRIM: R50.1
Unconnected: U1.7(NC)

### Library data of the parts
C1 C3 C35 C45 = rcl:C-EU: CAPACITOR, European symbol; MOUSER_OC: 81-GRM155R61A105KE15; MPN: GRM155R61A105KE15D; SUPPLIER: MURATA
C2 C4 C5 C7 C34 C44 = rcl:C-EU: CAPACITOR, European symbol
C31 C36 C41 C46 = rcl:C-EU: CAPACITOR, European symbol; VOLT: 100V
C32 C42 = rcl:C-EU: CAPACITOR, European symbol; TOL: 1%
C33 C43 = rcl:C-EU: CAPACITOR, European symbol; OC_FARNELL: 2611896; TOL: 1%
D31 D41 = UA_v2:DB3S308F; IMAX: 75mA; MPN: DB3S308F0L; OC_FARNELL: 2284977; SUPPLIER: PANASONIC
R1 R34-R36 R38 R39 R44-R46 R48-R51 R61 = rcl:R-EU_: RESISTOR, European symbol
R31-R33 R41-R43 = rcl:R-EU_: RESISTOR, European symbol; TOL: 0.1
R37 R47 = rcl:R-EU_: RESISTOR, European symbol; OC_FARNELL: 1811349; TOL: 0.1%
U1 = ua_cmp:AD8132ARZ: Low Cost, High Speed Differential Amplifier; ALTMPN: AD8132WARMZ; MPN: AD8132ARMZ; OC_FARNELL: 1660958; PACKAGE: MSOP8; SUPPLIER: AD

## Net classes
1 HV: clearance 0.203 mm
